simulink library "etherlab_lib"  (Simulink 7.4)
settings: Solver=ode45  SolverMode=SingleTasking  StartTime=0.0  StopTime=10.0  RelTol=1e-3
undefined symbols (not defined in the file or in its folder): ATD4, baumer_ecatencoder, bits, Boolean, BT, CoE, CW, DC, DI8DO8, Disabled, EK1100, EK1914, ekxxxx, EL1004, EL1262, EL1904, el1xxx, EL2004, EL2262, EL2535, el2535, EL2904, el2xxx, EL3002, EL3102, EL3201, EL3204, el320x_1, EL3255, EL3314, el331x, EL3356, el3356, EL3403, el3403, EL3602, el36x2, EL3702, el37x2, EL4002, el4xxx, EL5001, el500x, EL5021, el5021, EL5101, EL5152, El5152, EL51x1, el51xx, EL6001, el60xx, EL9110, el9xxx, EP1008, ep1xxx, EP2001, ep2xxx, EP3174, EP3182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
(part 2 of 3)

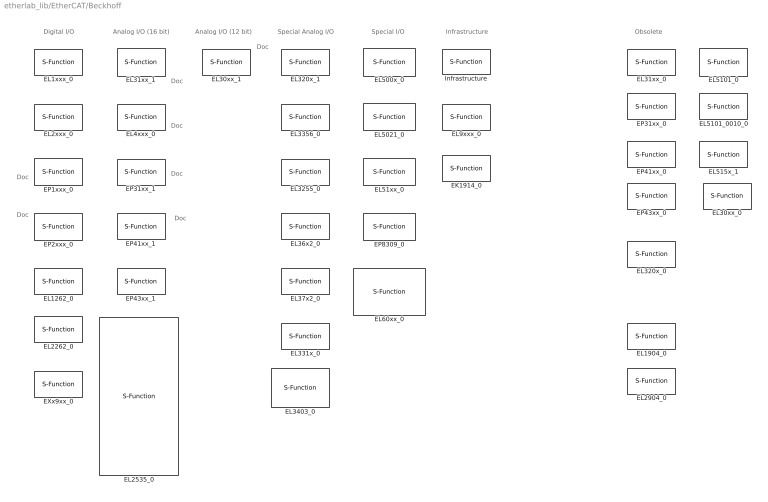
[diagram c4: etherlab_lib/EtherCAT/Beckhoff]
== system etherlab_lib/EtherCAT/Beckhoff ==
  note: Analog I/O (16 bit)
  note: Digital I/O
  note: Analog I/O (12 bit)
  note: Special Analog I/O
  note: Special I/O
  note: Infrastructure
  note: Obsolete
  note: Doc
  note: Doc
  note: Doc
  note: Doc
  note: Doc
  note: Doc
  note: Doc
  EK1914_0 : S-Function  FunctionName=ec_slave3  Parameters=Address,rv.SlaveConfig,rv.PortConfig,debug,tsample  SFunctionModules='ecrt_support'  EnableBusSupport=off  mask(EK1904){master=0, index=1, model=EK1914, stdio=on, safeio=off, tsample=-1, revision=, debug=}
      mask prompts: index "Slave Index"; model "Device Model"; stdio "Standard IO"; safeio "Safe IO"; tsample "Sample Time (-1 for inherited)"
      mask help: Beckhoff EtherCAT SAFE digital input/output coupler
      mask init:
      | Address = EtherCATSlave.formatAddress(master,index,tsample);
      | 
      | rv = ek1914(stdio, safeio);
      | 
      | rv.PortConfig.swap_io = EtherCATSlave.shouldSwapIoPorts();
      | 
      | text = sprintf('%s\\nM:%i Idx:%s', model, master, mat2str(index));
      | if numel(rv.PortConfig.input) > 1 || numel(rv.PortConfig.output) > 1
      |     EtherCATSlave.setPortNames(...
      |         {rv.PortConfig.input.portname},...
      |         {rv.PortConfig.output.portname});
      | 
      |     set_param(gcbh,'AttributesFormatString',text);
      | else
      |     set_param(gcbh,'AttributesFormatString','');
      |     set_param(gcbh,'MaskDisplay', strcat('disp(''',text,''')'));
      | end
  EL1262_0 : S-Function  FunctionName=ec_slave3  Parameters=Address,rv.SlaveConfig,rv.PortConfig,debug,tsample  SFunctionModules='ecrt_support'  EnableBusSupport=off  mask(EL1262){master=0, index=1, model=EL1262, one_ch=on, tsample=0, debug=0, revision=, dc_mode=10, dc_assign_activate=hex2dec('730'), dc_cycle0=0, dc_cycle0_factor=-10, dc_shift0=-10000, dc_shift0_factor=1, dc_shift0_input=off, dc_cycle1=0, dc_cycle1_factor=-1, dc_shift1=0, dc_shift1_factor=0}
      mask prompts: index "Slave Index"; model "Device Model"; one_ch "1 Ch. only"; tsample "Sample Time"; dc_mode "Mode/Oversampling"; dc_assign_activate "Assign Activate"; dc_cycle0 "Cycle Time Sync 0 [ns]"; dc_cycle0_factor "Factor"; dc_shift0 "Shift Time Sync0 [ns]"; dc_shift0_factor "Factor"; dc_shift0_input "Shift Time0 Input"; dc_cycle1 "Cycle Time Sync1 [ns]"; dc_cycle1_factor "Factor"; dc_shift1 "Shift Time Sync1 [ns]"; dc_shift1_factor "Factor"
      mask help: Beckhoff oversampling digital input
      mask init:
      | Address = EtherCATSlave.formatAddress(master,index,tsample);
      | 
      | rv = el1262(model).configure(one_ch,...
      |     [dc_mode, dc_assign_activate, ...
      |     dc_cycle0, dc_cycle0_factor,...
      |     dc_shift0, dc_shift0_factor, dc_shift0_input,...
      |     dc_cycle1, dc_cycle1_factor,...
      |     dc_shift1, dc_shift1_factor]);
      | rv.PortConfig.swap_io = EtherCATSlave.shouldSwapIoPorts();
  EL1904_0 : S-Function  FunctionName=ec_slave3  Parameters=Address,rv.SlaveConfig,rv.PortConfig,debug,tsample  SFunctionModules='ecrt_support'  EnableBusSupport=off  mask(EL1904){master=0, index=1, model=EL1904, safein=off, tsample=-1, revision=, debug=}
      mask prompts: index "Slave Index"; model "Device Model"; safein "Safe inputs"; tsample "Sample Time (-1 for inherited)"
      mask help: Beckhoff EtherCAT SAFE digital input
      mask init:
      | Address = EtherCATSlave.formatAddress(master,index,tsample);
      | 
      | rv = el1904(safein);
      | rv.PortConfig.swap_io = EtherCATSlave.shouldSwapIoPorts();
  EL1xxx_0 : S-Function  LoadFcn=el1xxx().checkModelName  FunctionName=ec_slave3  Parameters=Address,rv.SlaveConfig,rv.PortConfig,debug,tsample  SFunctionModules='ecrt_support'  EnableBusSupport=off  mask(EL1xxx){master=0, index=1, model=EL1004, revision=, vector=on, tsample=0, debug=0}
      mask prompts: index "Slave Index"; model "Device Model"; vector "Vector Outputs"; tsample "Sample Time"; debug "Debug Level"
      mask help: Beckhoff EtherCAT Digital Input
      mask init:
      | Address = EtherCATSlave.formatAddress(master,index,tsample);
      | 
      | rv = el1xxx(model).configure(vector);
      | rv.PortConfig.swap_io = EtherCATSlave.shouldSwapIoPorts();
  EL2262_0 : S-Function  FunctionName=ec_slave3  Parameters=Address,rv.SlaveConfig,rv.PortConfig,debug,tsample  SFunctionModules='ecrt_support'  EnableBusSupport=off  mask(EL2262){master=0, index=1, model=EL2262, one_ch=on, tsample=0, debug=0, revision=, dc_mode=10, dc_assign_activate=hex2dec('730'), dc_cycle0=0, dc_cycle0_factor=-10, dc_shift0=-10000, dc_shift0_factor=1, dc_shift0_input=off, dc_cycle1=0, dc_cycle1_factor=-1, dc_shift1=0, dc_shift1_factor=0}
      mask prompts: index "Slave Index"; model "Device Model"; one_ch "1 Ch. only"; tsample "Sample Time"; dc_mode "Mode/Oversampling"; dc_assign_activate "Assign Activate"; dc_cycle0 "Cycle Time Sync 0 [ns]"; dc_cycle0_factor "Factor"; dc_shift0 "Shift Time Sync0 [ns]"; dc_shift0_factor "Factor"; dc_shift0_input "Shift Time0 Input"; dc_cycle1 "Cycle Time Sync1 [ns]"; dc_cycle1_factor "Factor"; dc_shift1 "Shift Time Sync1 [ns]"; dc_shift1_factor "Factor"
      mask help: Beckhoff oversampling digital output
      mask init:
      | Address = EtherCATSlave.formatAddress(master,index,tsample);
      | 
      | rv = el2262(model).configure(one_ch,...
      |     [dc_mode, dc_assign_activate, ...
      |     dc_cycle0, dc_cycle0_factor,...
      |     dc_shift0, dc_shift0_factor, dc_shift0_input,...
      |     dc_cycle1, dc_cycle1_factor,...
      |     dc_shift1, dc_shift1_factor]);
      | rv.PortConfig.swap_io = EtherCATSlave.shouldSwapIoPorts();
  EL2535_0 : S-Function  LoadFcn=el2535().checkModelName  FunctionName=ec_slave3  Parameters=Address,rv.SlaveConfig,rv.PortConfig,debug,tsample  SFunctionModules='ecrt_support'  EnableBusSupport=off  mask(EL2535){master=0, index=1, model=EL2535, revision=, vector=on, tsample=0, debug=0, ch1enable=on, sdo_8=100, sdo_2=off, sdo_3=Default Value (see below), sdo_6=0, sdo_7=65535, sdo_9=350, sdo_10=6, sdo_11=50, sdo_1=off, sdo_12=100, sdo_13=10, ch2enable=on, sdo_23=100, sdo_17=off, sdo_18=Default Value (see below), sdo_21=0, sdo_22=65535, sdo_24=350, sdo_25=6, sdo_26=50, sdo_16=off, sdo_27=100, sdo_28=10, extra_output_1=None, extra_output_2=None, extra_output_3=None, extra_output_4=None}
      mask prompts: index "Slave Index"; model "Device Model"; vector "Vector Outputs"; tsample "Sample Time"; debug "Debug Level"; ch1enable "Enable"; sdo_8 "8000:10 - Maximum Current [%]"; sdo_2 "8000:04 - Invert Polarity"; sdo_3 "8000:05 - Watchdog"; sdo_6 "8000:0D - Default Output Value"; sdo_7 "8000:0E - Default Output Ramp"; sdo_9 "8000:12 - Current controller Kp"; sdo_10 "8000:13 - Current controller Ki"; sdo_11 "8000:14 - Current controller Kd"; sdo_1 "8000:03 - Enable dithering"; sdo_12 "8000:1E - Dithering Frequency [Hz]"; sdo_13 "8000:1F - Dithering Amplitude [% of max current in 8000:10]"; ch2enable "Enable"; sdo_23 "8010:10 - Maximum Current [%]"; sdo_17 "8010:04 - Invert Polarity"; sdo_18 "8010:05 - Watchdog"; sdo_21 "8010:0D - Default Output Value"; sdo_22 "8010:0E - Default Output Ramp"; sdo_24 "8010:12 - Current controller Kp"; sdo_25 "8010:13 - Current controller Ki"; sdo_26 "8010:14 - Current controller Kd"; sdo_16 "8010:03 - Enable dithering"; sdo_27 "8010:1E - Dithering Frequency [Hz]"; sdo_28 "8010:1F - Dithering Amplitude [% of max current in 8010:10]"; extra_output_1 "8000:21 - Extra Output 1"; extra_output_2 "8000:22 - Extra Output 2"; extra_output_3 "8010:21 - Extra Output 3"; extra_output_4 "8010:22 - Extra Output 4"
      mask help: Beckhoff EtherCAT PWM Output
      mask init:
      | Address = EtherCATSlave.formatAddress(master,index,tsample);
      | 
      | extra_output = [...
      |     extra_output_1,
      |     extra_output_2,
      |     extra_output_3,
      |     extra_output_4,
      | ];
      | channels = [ ...
      |     ch1enable; ...
      |     ch2enable; ...
      | ];
      | 
      |  sdo_4 = 0;
      |  sdo_5 = 65536;
      | sdo_19 = 0;
      | sdo_20 = 65536;
      | 
      | sdo_14 = el2535.extra_output_popup_sdo_map(extra_output_1);
      | sdo_15 = el2535.extra_output_popup_sdo_map(extra_output_2);
      | sdo_29 = el2535.extra_output_popup_sdo_map(extra_output_3);
      | sdo_30 = el2535.extra_output_popup_sdo_map(extra_output_4);
      | 
      | % fix watchdog value
      | sdo_3  =  sdo_3 - 1;
      | sdo_18 = sdo_18 - 1;
      | 
      | 
      | rv = el2535(model).configure(channels,extra_output, ...
      |     [  sdo_1,  sdo_2,  sdo_3,  sdo_4,  sdo_5,  sdo_6, ...
      |        sdo_7,  sdo_8,  sdo_9, sdo_10, sdo_11, sdo_12, ...
      |       sdo_13, sdo_14, sdo_15, sdo_16, sdo_17, sdo_18, ...
      |       sdo_19, sdo_20, sdo_21, sdo_22, sdo_23, sdo_24, ...
      |       sdo_25, sdo_26, sdo_27, sdo_28, sdo_29, sdo_30, ...
      |     ]);
      | 
      | rv.PortConfig.swap_io = EtherCATSlave.shouldSwapIoPorts();
      | 
      | inp = arrayfun(@(x) x.portname, rv.PortConfig.input, 'UniformOutput', false);
      | outp = arrayfun(@(x) x.portname, rv.PortConfig.output, 'UniformOutput', false);
      | 
      | if rv.OutputAmpere >= 1.0
      |     extra = sprintf('%s: %0.0f A', model, rv.OutputAmpere);
      | else
      |     extra = sprintf('%s: %0.0f mA', model, rv.OutputAmpere * 1000);
      | end
      | 
      | 
      | 
      | EtherCATSlave.setPortNames(inp, outp, extra);
      | 
      | set_param(gcb,'AttributesFormatString',...
      |     sprintf('%s\nM:%i Idx:%s',...
      |             extra,master,mat2str(index)))
  EL2904_0 : S-Function  FunctionName=ec_slave3  Parameters=Address,rv.SlaveConfig,rv.PortConfig,debug,tsample  SFunctionModules='ecrt_support'  EnableBusSupport=off  mask(EL2904){master=0, index=1, model=EL2904, safeout=off, tsample=-1, revision=, debug=}
      mask prompts: index "Slave Index"; model "Device Model"; safeout "Safe outputs"; tsample "Sample Time (-1 for inherited)"
      mask help: Beckhoff EtherCAT SAFE digital output
      mask init:
      | Address = EtherCATSlave.formatAddress(master,index,tsample);
      | 
      | rv = el2904(safeout);
      | rv.PortConfig.swap_io = EtherCATSlave.shouldSwapIoPorts();
  EL2xxx_0 : S-Function  LoadFcn=el2xxx().checkModelName  FunctionName=ec_slave3  Parameters=Address,rv.SlaveConfig,rv.PortConfig,debug,tsample  SFunctionModules='ecrt_support'  EnableBusSupport=off  mask(EL2xxx){master=0, index=1, model=EL2004, revision=, vector=on, diag=off, tsample=-1, debug=0}
      mask prompts: index "Slave Index"; model "Device Model"; vector "Vector Inputs"; diag "Diag Port"; tsample "Sample Time (-1 for inherited)"
      mask help: Beckhoff EtherCAT Digital Output
      mask init:
      | Address = EtherCATSlave.formatAddress(master,index,tsample);
      | 
      | rv = el2xxx(model).configure(vector,diag);
      | rv.PortConfig.swap_io = EtherCATSlave.shouldSwapIoPorts();
  EL30xx_0 : S-Function  LoadFcn=|  FunctionName=ec_slave3  Parameters=Address,rv.SlaveConfig,rv.PortConfig,debug,tsample  SFunctionModules='ecrt_support'  EnableBusSupport=off  mask(EL30xx){master=0, index=1, model=EL3002, vector=on, raw=off, scale=, offset=, tau=, tsample=0, debug=0}
      | el30xx('check')
      | if ~strcmp(bdroot(gcb),'etherlab_lib')
      |   disp([gcb ' is obsolete. Please replace'])
      | end
      mask prompts: index "Slave Index"; model "Device Model"; vector "Vector Output"; raw "Raw Bits"; scale "Output Scale"; offset "Output Offset"; tau "LPF Time Constant (sec)"; tsample "Sample Time"
      mask help: Beckhoff 1,2,4,8-Channel 16-Bit Analog Input
      mask init:
      | Address = EtherCATSlave.formatAddress(master,index,tsample);
      | 
      | el30xx('set');
      | 
      | rv = get_param(gcbh, 'UserData');
      | 
      | rv.PortConfig.swap_io = EtherCATSlave.shouldSwapIoPorts();
  EL30xx_1 : S-Function  LoadFcn=|  FunctionName=ec_slave3  Parameters=Address,rv.SlaveConfig,rv.PortConfig,debug,tsample  SFunctionModules='ecrt_support'  EnableBusSupport=off  mask(EL30xx){master=0, index=1, model=EL3002, revision=, vector=on, status=off, gain=[], offset=[], tau=[], tsample=0, debug=0, omega=, filter=Off, opmode=FreeRun, fastop=off}
      | el30xx_1().checkModelName()
      | EtherCATSlave.checkFilter()
      mask prompts: index "Slave Index"; model "Device Model"; vector "Vector Output"; status "Status Output"; gain "Output Scale"; offset "Output Offset"; tau "LPF time constant (s)"; tsample "Sample Time"; omega "deprecated"; opmode "Synchronization Mode (1C33:01.0)"; fastop "FastOp Mode (1C33:01.15)"
      mask help: Beckhoff 1,2,4,8-Channel 16-Bit Analog Input
      mask init:
      | Address = EtherCATSlave.formatAddress(master,index,tsample);
      | 
      | rv = el30xx_1(model).configure(status,vector,...
      |     EtherCATSlave.configureScale(2^15,gain,offset,tau),...
      |     [filter,opmode,fastop]);
      | 
      | rv.PortConfig.swap_io = EtherCATSlave.shouldSwapIoPorts();
      | 
      | if vector
      |     set_param(gcb,'AttributesFormatString','');
      | 
      |     set_param(gcb,'MaskDisplay',...
      |         sprintf('disp(''%s %s\\nM:%i Idx:%s'')',...
      |         model,rv.function,master,mat2str(index)))
      | else
      |     EtherCATSlave.setPortNames({},...
      |         {rv.PortConfig.output.portname})
      |     
      |     set_param(gcb,'AttributesFormatString',...
      |         sprintf('%s %s\nM:%i Idx:%s',...
      |         model,rv.function,master,mat2str(index)))
      | end
  EL31xx_0 : S-Function  LoadFcn=|  FunctionName=ec_slave3  Parameters=Address,rv.SlaveConfig,rv.PortConfig,debug,tsample  SFunctionModules='ecrt_support'  EnableBusSupport=off  mask(EL31xx){master=0, index=1, model=EL3102, dc=DC-Synchron, vector=on, raw=off, scale=, offset=, tau=, tsample=0, debug=0}
      | el31xx('check')
      | if ~strcmp(bdroot(gcb),'etherlab_lib')
      |   disp([gcb ' is obsolete. Please replace'])
      | end
      mask prompts: index "Slave Index"; model "Device Model"; dc "Distributed Clock"; vector "Vector Output"; raw "Raw output"; scale "Output Scale"; offset "Output Offset"; tau "LPF Time Constant (sec)"; tsample "Sample Time"
      mask help: Beckhoff 2,4,8-Channel 16-Bit Analog Input with Distributed Clocks Status output is not supported
      mask init:
      | Address = EtherCATSlave.formatAddress(master,index,tsample);
      | 
      | el31xx('set');  % Report errors
      | 
      | rv = get_param(gcb,'UserData');
      | rv.PortConfig.swap_io = EtherCATSlave.shouldSwapIoPorts();
  EL31xx_1 : S-Function  LoadFcn=|  FunctionName=ec_slave3  Parameters=Address,rv.SlaveConfig,rv.PortConfig,debug,tsample  SFunctionModules='ecrt_support'  EnableBusSupport=off  mask(EL31xx){master=0, index=1, model=EL3102, revision=, vector=on, status=off, filter=Off, gain=[], offset=[], tau=[], tsample=0, debug=0, omega=, dc_mode=Free Run/SM-Synchron, dc_assign_activate=hex2dec('700'), dc_cycle0=[], dc_cycle0_factor=[], dc_shift0=[], dc_shift0_factor=[], dc_shift0_input=off, dc_cycle1=[], dc_cycle1_factor=[], dc_shift1=[], dc_shift1_factor=[]}
      | el31xx_1().checkModelName()
      | EtherCATSlave.checkFilter()
      mask prompts: index "Slave Index"; model "Device Model"; vector "Vector Output"; status "Status output"; gain "Output Gain"; offset "Output Offset"; tau "LPF time constant (s)"; tsample "Sample Time"; omega "deprecated"; dc_mode "Mode"; dc_assign_activate "Assign Activate"; dc_cycle0 "Cycle Time Sync 0"; dc_cycle0_factor "Factor"; dc_shift0 "Shift Time Sync0"; dc_shift0_factor "Factor"; dc_shift0_input "Shift Time0 Input"; dc_cycle1 "Cycle Time Sync1"; dc_cycle1_factor "Factor"; dc_shift1 "Shift Time Sync1"; dc_shift1_factor "Factor"
      mask help: Beckhoff 2,4,8-Channel 16-Bit Analog Input with Distributed Clocks
      mask init:
      | Address = EtherCATSlave.formatAddress(master,index,tsample);
      | 
      | rv = el31xx_1(model).configure(status,vector,...
      |     EtherCATSlave.configureScale(2^15,gain,offset,tau),...
      |     [dc_mode, dc_assign_activate, ...
      |      dc_cycle0, dc_cycle0_factor, ...
      |      dc_shift0, dc_shift0_factor, dc_shift0_input, ...
      |      dc_cycle1, dc_cycle1_factor, ...
      |      dc_shift1, dc_shift1_factor], ...
      |      filter);
      | 
      | rv.PortConfig.swap_io = EtherCATSlave.shouldSwapIoPorts();
      | 
      | if vector || model(6) == '1'
      |     set_param(gcb,'AttributesFormatString','');
      | 
      |     set_param(gcb,'MaskDisplay',...
      |         sprintf('disp(''%s\\nM:%i Idx:%s'')',...
      |         model,master,mat2str(index)))
      | else
      |     EtherCATSlave.setPortNames({},...
      |         {rv.PortConfig.output.portname})
      |     
      |     set_param(gcb,'AttributesFormatString',...
      |         sprintf('%s\nM:%i Idx:%s',...
      |         model,master,mat2str(index)))
      | end
  EL320x_0 : S-Function  LoadFcn=|  FunctionName=ec_slave3  Parameters=Address,rv.SlaveConfig,rv.PortConfig,debug,tsample  SFunctionModules='ecrt_support'  EnableBusSupport=off  mask(EL320x){master=0, index=1, model=EL3204, rtd=0, technology=2, filter=50 Hz, vector=on, enable_status=on, tsample=0, debug=0}
      | el320x('check')
      | if ~strcmp(bdroot(gcb),'etherlab_lib')
      |   disp([gcb ' is obsolete. Please replace'])
      | end
      mask prompts: index "Slave Index"; model "Device Model"; rtd "RTD-Element (CoE 80x0:19)"; technology "Connection Technology (CoE 80x0:1A)"; filter "Filter (CoE 8000:15)"; vector "Vector Output"; enable_status "Status Port"; tsample "Sample Time"
      mask help: Beckhoff 1, 2, 4-Channel Input Terminal Pt100 (RTD)
      mask init:
      | Address = EtherCATSlave.formatAddress(master,index,tsample);
      | 
      | SdoConfig = [];
      | 
      | rv = get_param(gcbh,'UserData');
      | 
      | count = numel(rv.SlaveConfig.sm{1}{3});
      | 
      | err = {};
      | if numel(rtd) == 1
      |     rtd = repmat(rtd,1,count);
      | elseif numel(rtd) ~= count
      |     err = {['- Mask option "RTD Element"' ...
      |         ' is not a scalar or vector with ' ...
      |         num2str(count) ' elements']};
      | end
      | 
      | if numel(technology) == 1
      |     technology = repmat(technology,1,count);
      | elseif numel(technology) ~= count
      |     err = horzcat(err, ['- Mask option "Connection Technology"' ...
      |         ' is not a scalar or vector with ' ...
      |         num2str(count) ' elements']);
      | end
      | 
      | if ~isempty(err)
      |     errordlg(err,gcb);
      |     return
      | end
      | 
      | rv.SlaveConfig.sdo = num2cell(vertcat(...
      |     [hex2dec('8000'),6,8,1],...
      |     [hex2dec('8000'),hex2dec('15'),16,filter+1],...
      |     horzcat(repmat(hex2dec('8000') + 16*(0:count-1)',2,1),...
      |             [hex2dec('19')*ones(count,1);hex2dec('1a')*ones(count,1)],...
      |             16*ones(count*2,1),...
      |             vertcat(reshape(rtd,[],1),...
      |                     reshape(technology,[],1)))));
      | 
      | rv.PortConfig.swap_io = EtherCATSlave.shouldSwapIoPorts();
  EL320x_1 : S-Function  LoadFcn=el320x_1().checkModelName()  FunctionName=ec_slave3  Parameters=Address,rv.SlaveConfig,rv.PortConfig,debug,tsample  SFunctionModules='ecrt_support'  EnableBusSupport=off  mask(EL320x){master=0, index=1, model=EL3201, revision=, filter=Off, vector=on, status=off, tsample=0, debug=0, sdo_01=Pt100 -200...850C, sdo_02=2-wire, sdo_03=0, sdo_04=Pt100 -200...850C, sdo_05=2-wire, sdo_06=0, sdo_07=Pt100 -200...850C, sdo_08=2-wire, sdo_09=0, sdo_10=Pt100 -200...850C, sdo_11=2-wire, sdo_12=0, sdo_13=Pt100 -200...850C, sdo_14=2-wire, sdo_15=0, sdo_16=Pt100 -200...850C, sdo_17=2-wire, sdo_18=0, sdo_19=Pt100 -200...850C, sdo_20=2-wire, sdo_21=0, sdo_22=Pt100 -200...850C, sdo_23=2-wire, sdo_24=0}
      mask prompts: index "Slave Index"; model "Device Model"; vector "Vector Output"; status "Status Port"; tsample "Sample Time"; sdo_01 "RTD-Element"; sdo_02 "Technology"; sdo_03 "Wire Calibration (1/32 Ohm)"; sdo_04 "RTD-Element"; sdo_05 "Technology"; sdo_06 "Wire Calibration (1/32 Ohm)"; sdo_07 "RTD-Element"; sdo_08 "Technology"; sdo_09 "Wire Calibration (1/32 Ohm)"; sdo_10 "RTD-Element"; sdo_11 "Technology"; sdo_12 "Wire Calibration (1/32 Ohm)"; sdo_13 "RTD-Element"; sdo_14 "Technology"; sdo_15 "Wire Calibration (1/32 Ohm)"; sdo_16 "RTD-Element"; sdo_17 "Technology"; sdo_18 "Wire Calibration (1/32 Ohm)"; sdo_19 "RTD-Element"; sdo_20 "Technology"; sdo_21 "Wire Calibration (1/32 Ohm)"; sdo_22 "RTD-Element"; sdo_23 "Technology"; sdo_24 "Wire Calibration (1/32 Ohm)"
      mask help: Beckhoff 1, 2, 4-Channel Input Terminal Pt100 (RTD)
      mask init:
      | Address = EtherCATSlave.formatAddress(master,index,tsample);
      | 
      | rv = el320x_1(model).configure(status,vector,filter,...
      |     [sdo_01,sdo_04,sdo_07,sdo_10,sdo_13,sdo_16,sdo_19,sdo_22] - 1,...
      |     [sdo_02,sdo_05,sdo_08,sdo_11,sdo_14,sdo_17,sdo_20,sdo_23] - 1,...
      |     [sdo_03,sdo_06,sdo_09,sdo_12,sdo_15,sdo_18,sdo_21,sdo_24]);
      | 
      | rv.PortConfig.swap_io = EtherCATSlave.shouldSwapIoPorts();
      | 
      | if vector || model(6) == '1'
      |     set_param(gcb,'AttributesFormatString','');
      | 
      |     set_param(gcb,'MaskDisplay',...
      |         sprintf('disp(''%s\\nM:%i Idx:%s'')',...
      |         model,master,mat2str(index)))
      | else
      |     EtherCATSlave.setPortNames({},...
      |         {rv.PortConfig.output.portname})
      |     
      |     set_param(gcb,'AttributesFormatString',...
      |         sprintf('%s\nM:%i Idx:%s',...
      |         model,master,mat2str(index)))
      | end
  EL3255_0 : S-Function  LoadFcn=|  FunctionName=ec_slave3  Parameters=Address,rv.SlaveConfig,rv.PortConfig,debug,tsample  SFunctionModules='ecrt_support'  EnableBusSupport=off  mask(EL3255){master=0, index=1, model=EL3255, revision=, channels=1, vector=off, gain=[], offset=[], tau=[], tsample=0, debug=0, omega=, dc_mode=Free Run/SM-Synchron, dc_assign_activate=hex2dec('700'), dc_cycle0=[], dc_cycle0_factor=[], dc_shift0=[], dc_shift0_factor=[], dc_shift0_input=off, dc_cycle1=[], dc_cycle1_factor=[], dc_shift1=[], dc_shift1_factor=[], sdo_01=off, sdo_02=50 Hz, sdo_03=Off (up to 10 kOhm), sdo_04=Off (up to 10 kOhm), sdo_05=Off (up to 10 kOhm), sdo_06=Off (up to 10 kOhm), sdo_07=Off (up to 10 kOhm)}
      | el3255().checkModelName()
      | EtherCATSlave.checkFilter
      mask prompts: index "Slave Index"; model "Device Model"; channels "Active Channels"; vector "Vector Outputs"; tau "LPF time constant (s)"; tsample "Sample Time"; debug "Debug Level"; omega "deprecated"; dc_mode "Distributed Clock"; dc_assign_activate "Assign Activate"; dc_cycle0 "Cycle Time Sync 0"; dc_cycle0_factor "Factor"; dc_shift0 "Shift Time Sync0"; dc_shift0_factor "Factor"; dc_shift0_input "Shift Time0 Input"; dc_cycle1 "Cycle Time Sync1"; dc_cycle1_factor "Factor"; dc_shift1 "Shift Time Sync1"; dc_shift1_factor "Factor"; sdo_01 "Enable Filter (#x8000:06)"; sdo_02 "Filter settings (#x8000:15)"; sdo_03 "Load resistance 1"; sdo_04 "Load resistance 2"; sdo_05 "Load resistance 3"; sdo_06 "Load resistance 4"; sdo_07 "Load resistance 5"
      mask help: Beckhoff EtherCAT 5Ch. potentiometer measurement with sensor supply
      mask init:
      | Address = EtherCATSlave.formatAddress(master,index,tsample);
      | 
      | rv = el3255(model).configure(channels,vector,...
      |     [dc_mode, dc_assign_activate, ...
      |     dc_cycle0, dc_cycle0_factor,...
      |     dc_shift0, dc_shift0_factor, dc_shift0_input,...
      |     dc_cycle1, dc_cycle1_factor,...
      |     dc_shift1, dc_shift1_factor], ...
      |     EtherCATSlave.configureScale(2^15,gain,offset,tau),...
      |     [sdo_01, ...
      |      [sdo_02, sdo_03, sdo_04, sdo_05, sdo_06, sdo_07]-1]);
      | 
      | rv.PortConfig.swap_io = EtherCATSlave.shouldSwapIoPorts();
  EL331x_0 : S-Function  LoadFcn=el331x().checkModelName  FunctionName=ec_slave3  Parameters=Address,rv.SlaveConfig,rv.PortConfig,debug,tsample  SFunctionModules='ecrt_support'  EnableBusSupport=off  mask(EL331x){master=0, index=1, model=EL3314, revision=, vector=on, status=off, tsample=0, debug=0, sdo_8000_02=0.1, sdo_8000_0C=Internal, sdo_8000_15=50 Hz, sdo_8000_19=0: Type K, sdo_8000_1A=Inactive, sdo_8010_02=0.1, sdo_8010_0C=Internal, sdo_8010_15=50 Hz, sdo_8010_19=0: Type K, sdo_8010_1A=Inactive, sdo_8020_02=0.1, sdo_8020_0C=Internal, sdo_8020_15=50 Hz, sdo_8020_19=0: Type K, sdo_8020_1A=Inactive, sdo_8030_02=0.1, sdo_8030_0C=Internal, sdo_8030_15=50 Hz, sdo_8030_19=0: Type K, sdo_8030_1A=Inactive, sdo_8040_02=0.1, sdo_8040_0C=Internal, sdo_8040_15=50 Hz, sdo_8040_19=0: Type K, sdo_8040_1A=Inactive, sdo_8050_02=0.1, sdo_8050_0C=Internal, sdo_8050_15=50 Hz, sdo_8050_19=0: Type K, sdo_8050_1A=Inactive, sdo_8060_02=0.1, sdo_8060_0C=Internal, sdo_8060_15=50 Hz, sdo_8060_19=0: Type K, sdo_8060_1A=Inactive, sdo_8070_02=0.1, sdo_8070_0C=Internal, sdo_8070_15=50 Hz, sdo_8070_19=0: Type K, sdo_8070_1A=Inactive}
      mask prompts: index "Slave Index"; model "Device Model"; vector "Vector Outputs"; status "Status Output"; tsample "Sample Time"; sdo_8000_02 "Resolution (#x8000:02)"; sdo_8000_0C "Coldjunction Compensation (#x8000:0C)"; sdo_8000_15 "Filter settings (#x8000:15)"; sdo_8000_19 "TC Element (#x8000:19)"; sdo_8000_1A "MC Filter (#x8000:1A)"; sdo_8010_02 "Resolution (#x8010:02)"; sdo_8010_0C "Coldjunction Compensation (#x8010:0C)"; sdo_8010_15 "Filter settings (#x8010:15)"; sdo_8010_19 "TC Element (#x8010:19)"; sdo_8010_1A "MC Filter (#x8010:1A)"; sdo_8020_02 "Resolution (#x8020:02)"; sdo_8020_0C "Coldjunction Compensation (#x8020:0C)"; sdo_8020_15 "Filter settings (#x8020:15)"; sdo_8020_19 "TC Element (#x8020:19)"; sdo_8020_1A "MC Filter (#x8020:1A)"; sdo_8030_02 "Resolution (#x8030:02)"; sdo_8030_0C "Coldjunction Compensation (#x8030:0C)"; sdo_8030_15 "Filter settings (#x8030:15)"; sdo_8030_19 "TC Element (#x8030:19)"; sdo_8030_1A "MC Filter (#x8030:1A)"; sdo_8040_02 "Resolution (#x8040:02)"; sdo_8040_0C "Coldjunction Compensation (#x8040:0C)"; sdo_8040_15 "Filter settings (#x8040:15)"; sdo_8040_19 "TC Element (#x8040:19)"; sdo_8040_1A "MC Filter (#x8040:1A)"; sdo_8050_02 "Resolution (#x8050:02)"; sdo_8050_0C "Coldjunction Compensation (#x8050:0C)"; sdo_8050_15 "Filter settings (#x8050:15)"; sdo_8050_19 "TC Element (#x8050:19)"; sdo_8050_1A "MC Filter (#x8050:1A)"; sdo_8060_02 "Resolution (#x8060:02)"; sdo_8060_0C "Coldjunction Compensation (#x8060:0C)"; sdo_8060_15 "Filter settings (#x8060:15)"; sdo_8060_19 "TC Element (#x8060:19)"; sdo_8060_1A "MC Filter (#x8060:1A)"; sdo_8070_02 "Resolution (#x8070:02)"; sdo_8070_0C "Coldjunction Compensation (#x8070:0C)"; sdo_8070_15 "Filter settings (#x8070:15)"; sdo_8070_19 "TC Element (#x8070:19)"; sdo_8070_1A "MC Filter (#x8070:1A)"
      mask help: Beckhoff thermocouple input slave terminal
      mask init:
      | Address = EtherCATSlave.formatAddress(master,index,tsample);
      | 
      | rv = el331x(model).configure(vector,status,...
      |     [sdo_8000_02,sdo_8000_0C,sdo_8000_15,sdo_8000_19,sdo_8000_1A;
      |      sdo_8010_02,sdo_8010_0C,sdo_8010_15,sdo_8010_19,sdo_8010_1A;
      |      sdo_8020_02,sdo_8020_0C,sdo_8020_15,sdo_8020_19,sdo_8020_1A;
      |      sdo_8030_02,sdo_8030_0C,sdo_8030_15,sdo_8030_19,sdo_8030_1A;
      |      sdo_8040_02,sdo_8040_0C,sdo_8040_15,sdo_8040_19,sdo_8040_1A;
      |      sdo_8050_02,sdo_8050_0C,sdo_8050_15,sdo_8050_19,sdo_8050_1A;
      |      sdo_8060_02,sdo_8060_0C,sdo_8060_15,sdo_8060_19,sdo_8060_1A;
      |      sdo_8070_02,sdo_8070_0C,sdo_8070_15,sdo_8070_19,sdo_8070_1A]);
      | 
      | rv.PortConfig.swap_io = EtherCATSlave.shouldSwapIoPorts();
  EL3356_0 : S-Function  LoadFcn=el3356().checkModelName()  FunctionName=ec_slave3  Parameters=Address,rv.SlaveConfig,rv.PortConfig,debug,tsample  SFunctionModules='ecrt_support'  EnableBusSupport=off  mask(EL3356){master=0, index=1, model=EL3356, revision=, adc=off, range=[], scale=[], offset=[], tau=[], tsample=-1, debug=0, omega=, dc_mode=SM-Synchron, dc_assign_activate=hex2dec('320'), dc_cycle0=0, dc_cycle0_factor=1, dc_shift0=0, dc_shift0_factor=0, dc_shift0_input=off, dc_cycle1=0, dc_cycle1_factor=1, dc_shift1=0, dc_shift1_factor=0, sdo_01=off, sdo_02=off, sdo_03=on, sdo_04=on, sdo_05=off, sdo_06=FIR 50 Hz, sdo_07=FIR 50 Hz, sdo_08=10, sdo_09=20, sdo_10=1000, sdo_11=5, sdo_12=1800, sdo_13=10, sdo_14=off, sdo_15=50 Hz FIR, sdo_16=off, sdo_17=50 Hz FIR}
      mask prompts: index "Slave Index"; model "Device Model"; adc "2 ch ADC only"; range "RMB Range [mV/V]"; scale "Output Scale"; offset "Output Offset"; tau "LPF time constant (s)"; tsample "Sample Time"; omega "deprecated"; dc_mode "Mode"; dc_assign_activate "Assign Activate"; dc_cycle0 "Cycle Time Sync 0"; dc_cycle0_factor "Factor"; dc_shift0 "Shift Time Sync0"; dc_shift0_factor "Factor"; dc_shift0_input "Shift Time0 Input"; dc_cycle1 "Cycle Time Sync1"; dc_cycle1_factor "Factor"; dc_shift1 "Shift Time Sync1"; dc_shift1_factor "Factor"; sdo_01 "Mode 0 Enable Filter (#x8000:01)"; sdo_02 "Mode 1 Enable Filter (#x8000:02)"; sdo_03 "Mode 0 Enable Averager (#x8000:03)"; sdo_04 "Mode 1 Enable Averager (#x8000:04)"; sdo_05 "Symmetric Reference Potential (#x8000:05)"; sdo_06 "Mode 0 Filter (#x8000:11)"; sdo_07 "Mode 1 Filter (#x8000:12)"; sdo_08 "Dynamic filter change time [0.01s] (#x8000:13)"; sdo_09 "Dynamic filter delta (#x8000:14)"; sdo_10 "Steady state window (#x8000:29)"; sdo_11 "Steady state tolerance (#x8000:2a)"; sdo_12 "Calibration interval [100ms] (#x8000:31)"; sdo_13 "Test interval (#x8000:32)"; sdo_14 "Enable ch. 1 filter (#x8010:06)"; sdo_15 "Ch.1 filter settings (#x8010:15)"; sdo_16 "Enable ch.2 filter (#x8020:06)"; sdo_17 "Ch.2 filter settings (#x8020:15)"
      mask help: Beckhoff DMS Input with Distributed Clocks
      mask init:
      | Address = EtherCATSlave.formatAddress(master,index,tsample);
      | 
      | rv = el3356(model).configure(adc,range,...
      |     [dc_mode, dc_assign_activate, ...
      |     dc_cycle0, dc_cycle0_factor,...
      |     dc_shift0, dc_shift0_factor, dc_shift0_input,...
      |     dc_cycle1, dc_cycle1_factor,...
      |     dc_shift1, dc_shift1_factor], ...
      |     EtherCATSlave.configureScale(2^31,scale,offset,tau),...
      |     [sdo_01,   sdo_02,   sdo_03, sdo_04, sdo_05, ...
      |      sdo_06-1, sdo_07-1, sdo_08, sdo_09, sdo_10, ...
      |      sdo_11,   sdo_12,   sdo_13, ...
      |      sdo_14,   sdo_15-1, ...
      |      sdo_16,   sdo_17-1]);
      | 
      | rv.PortConfig.swap_io = EtherCATSlave.shouldSwapIoPorts();
      | 
      | EtherCATSlave.setPortNames(...
      |     {rv.PortConfig.input.portname},...
      |     {rv.PortConfig.output.portname});
      | 
      | set_param(gcb,'AttributesFormatString',...
      |     sprintf('%s\nM:%i Idx:%s',...
      |             model,master,mat2str(index)))
  EL3403_0 : S-Function  LoadFcn=el3403().checkModelName()  FunctionName=ec_slave3  Parameters=Address,rv.SlaveConfig,rv.PortConfig,debug,tsample  SFunctionModules='ecrt_support'  EnableBusSupport=off  mask(EL3403){master=0, index=1, model=EL3403, variant=off, current=1, voltage=1, tsample=-1, revision=[223031378 1441792], debug=0, freq=Phase L1, ref=Phase L1, zerocross=5, cycle=10}
      mask prompts: index "Slave Index"; model "Device Model"; variant "Variants"; current "Current Transformation Ratio 1:"; voltage "Voltage Transformation Ratio 1:"; tsample "Sample Time (-1 inherited)"; freq "Frequency channel (F800:05)"; ref "Reference channel (F800:0E)"; zerocross "Zero cross timeout (F800:21)"; cycle "Line cycle (F800:22)"
      mask help: Beckhoff 3-phase power measurement terminal
      mask init:
      | Address = EtherCATSlave.formatAddress(master,index,tsample);
      | 
      | rv = el3403(model).configure(variant,current,voltage,...
      |     [freq-1, ref-1, zerocross, cycle]);
      | 
      | rv.PortConfig.swap_io = EtherCATSlave.shouldSwapIoPorts();
      | 
      | EtherCATSlave.setPortNames(...
      |     {rv.PortConfig.input.portname},...
      |     {rv.PortConfig.output.portname});
      | 
      | set_param(gcb,'AttributesFormatString',...
      |     sprintf('%s\nM:%i Idx:%s',...
      |             model,master,mat2str(index)))
  EL36x2_0 : S-Function  LoadFcn=el36x2().checkModelName()  FunctionName=ec_slave3  Parameters=Address,rv.SlaveConfig,rv.PortConfig,debug,tsample,rv.Parameter,scale,offset  SFunctionModules='ecrt_support'  EnableBusSupport=off  mask(EL36x2){master=0, index=1, model=EL3602, revision=, vector=on, status=off, one_ch=on, scale=[], offset=[], tsample=0, debug=, sdo_x8000_15=50 Hz, sdo_x8000_19=+/- 10 V, sdo_x8010_19=+/- 10 V}
      mask prompts: index "Slave Index"; model "Device Model"; vector "Vector Output"; status "Status port"; one_ch "1 Ch. only"; scale "Output Scale"; offset "Output Offset"; tsample "Sample Time"; sdo_x8000_15 "Filter (#x8000:15)"; sdo_x8000_19 "Range Ch.1 (#x8000:19)"; sdo_x8010_19 "Range Ch.2 (#x8010:19)"
      mask help: Beckhoff 24-bit analog input terminal
      mask init:
      | Address = EtherCATSlave.formatAddress(master,index,tsample);
      | 
      | rv = el36x2(model).configure(one_ch,vector,status,...
      |     [numel(scale), 6; numel(offset), 7],...
      |     sdo_x8000_15-1,...
      |     [sdo_x8000_19,sdo_x8010_19]-1);
      | 
      | rv.PortConfig.swap_io = EtherCATSlave.shouldSwapIoPorts();
      | 
      | if ~status || vector || model(6) == '1' || one_ch
      |     set_param(gcb,'AttributesFormatString','');
      | 
      |     set_param(gcb,'MaskDisplay',...
      |         sprintf('disp(''%s\\nM:%i Idx:%s'')',...
      |         model,master,mat2str(index)))
      | else
      |     EtherCATSlave.setPortNames({},...
      |         {rv.PortConfig.output.portname})
      |     
      |     set_param(gcb,'AttributesFormatString',...
      |         sprintf('%s\nM:%i Idx:%s',...
      |         model,master,mat2str(index)))
      | end
  EL37x2_0 : S-Function  LoadFcn=el37x2().checkModelName()  FunctionName=ec_slave3  Parameters=Address,rv.SlaveConfig,rv.PortConfig,debug,tsample  SFunctionModules='ecrt_support'  EnableBusSupport=off  mask(EL37x2){master=0, index=1, model=EL3702, revision=, one_ch=off, scale=[], offset=[], tsample=0, debug=0, dc_mode=10, dc_assign_activate=hex2dec('730'), dc_cycle0=0, dc_cycle0_factor=-10     % 10-times OS, dc_shift0=-10000, dc_shift0_factor=1, dc_shift0_input=off, dc_cycle1=0, dc_cycle1_factor=-1, dc_shift1=0, dc_shift1_factor=0}
      mask prompts: index "Slave Index"; model "Device Model"; one_ch "1 Ch. only"; scale "Output Scale"; offset "Output Offset"; tsample "Sample Time"; dc_mode "Mode/Oversampling"; dc_assign_activate "Assign Activate"; dc_cycle0 "Cycle Time Sync 0 [ns]"; dc_cycle0_factor "Factor"; dc_shift0 "Shift Time Sync0 [ns]"; dc_shift0_factor "Factor"; dc_shift0_input "Shift Time0 Input"; dc_cycle1 "Cycle Time Sync1 [ns]"; dc_cycle1_factor "Factor"; dc_shift1 "Shift Time Sync1 [ns]"; dc_shift1_factor "Factor"
      mask help: Beckhoff oversampling analog input
      mask init:
      | Address = EtherCATSlave.formatAddress(master,index,tsample);
      | 
      | rv = el37x2(model).configure(one_ch,...
      |     [dc_mode, dc_assign_activate, ...
      |     dc_cycle0, dc_cycle0_factor,...
      |     dc_shift0, dc_shift0_factor, dc_shift0_input,...
      |     dc_cycle1, dc_cycle1_factor,...
      |     dc_shift1, dc_shift1_factor], ...
      |     EtherCATSlave.configureScale(2^15,scale,offset));
      | 
      | rv.PortConfig.swap_io = EtherCATSlave.shouldSwapIoPorts();
  EL4xxx_0 : S-Function  LoadFcn=el4xxx().checkModelName()  FunctionName=ec_slave3  Parameters=Address,rv.SlaveConfig,rv.PortConfig,debug,tsample  SFunctionModules='ecrt_support'  EnableBusSupport=off  mask(EL4xxx){master=0, index=1, model=EL4002, revision=, vector=on, scale=[], tsample=-1, debug=0, dc_mode=Free Run, dc_assign_activate=hex2dec('700'), dc_cycle0=0, dc_cycle0_factor=1, dc_shift0=0, dc_shift0_factor=0, dc_shift0_input=off, dc_cycle1=0, dc_cycle1_factor=1, dc_shift1=10000, dc_shift1_factor=0}
      mask prompts: index "Slave Index"; model "Device Model"; vector "Vector Input"; scale "Input Scale (empty for none)"; tsample "Sample Time (-1 for inherited)"; dc_mode "Distributed Clocks"; dc_assign_activate "Assign Activate"; dc_cycle0 "Cycle Time Sync 0"; dc_cycle0_factor "Factor"; dc_shift0 "Shift Time Sync0"; dc_shift0_factor "Factor"; dc_shift0_input "Shift Time0 Input"; dc_cycle1 "Cycle Time Sync1"; dc_cycle1_factor "Factor"; dc_shift1 "Shift Time Sync1"; dc_shift1_factor "Factor"
      mask help: Beckhoff Analog Output
      mask init:
      | Address = EtherCATSlave.formatAddress(master,index,tsample);
      | 
      | rv = el4xxx(model).configure(vector,...
      |     EtherCATSlave.configureScale(2^15,scale),...
      |     [dc_mode, dc_assign_activate,...
      |      dc_cycle0, dc_cycle0_factor,...
      |      dc_shift0, dc_shift0_factor, dc_shift0_input,...
      |      dc_cycle1, dc_cycle1_factor,...
      |      dc_shift1, dc_shift1_factor]);
      | 
      | rv.PortConfig.swap_io = EtherCATSlave.shouldSwapIoPorts();
  EL500x_0 : S-Function  LoadFcn=el500x().checkModelName()  FunctionName=ec_slave3  Parameters=Address,rv.SlaveConfig,rv.PortConfig,debug,tsample  SFunctionModules='ecrt_support'  EnableBusSupport=off  mask(EL500x){master=0, index=1, model=EL5001, revision=, pdo_x1A02=off, tsample=0, debug=0, dc_mode=FreeRun/SM-Synchron, dc_assign_activate=hex2dec('700')    % '120' for EL5001-0011, dc_cycle0=0, dc_cycle0_factor=1, dc_shift0=0, dc_shift0_factor=0, dc_shift0_input=off, dc_cycle1=0, dc_cycle1_factor=1, dc_shift1=15000, dc_shift1_factor=0, sdo_01=off, sdo_02=off, sdo_03=off, sdo_04=off, sdo_05=off, sdo_06=Gray, sdo_07=500k, sdo_08=Multiturn (25 bits), sdo_09=25, sdo_10=24, sdo_11=0, sdo_12=off, sdo_13=off, sdo_14=off, sdo_15=off, sdo_16=Gray, sdo_17=500k, sdo_18=Multiturn (25 bits), sdo_19=25, sdo_20=24, sdo_21=0}
      mask prompts: index "Slave Index"; model "Device Model"; pdo_x1A02 "Timestamp (PDO #x1a02)"; tsample "Sample Time"; dc_mode "DC Mode"; dc_assign_activate "Assign Activate"; dc_cycle0 "Cycle Time Sync 0 [ns]"; dc_cycle0_factor "Factor"; dc_shift0 "Shift Time Sync0 [ns]"; dc_shift0_factor "Factor"; dc_shift0_input "Shift Time0 Input"; dc_cycle1 "Cycle Time Sync1 [ns]"; dc_cycle1_factor "Factor"; dc_shift1 "Shift Time Sync1 [ns]"; dc_shift1_factor "Factor"; sdo_01 "8000:01 - Disable frame error"; sdo_02 "8000:02 - Enable power failure bit"; sdo_03 "8000:03 - Enable inhibit time"; sdo_04 "8000:04 - Enable test mode"; sdo_05 "8000:05 - Check SSI-frame size"; sdo_06 "8000:06 - SSI-coding"; sdo_07 "8000:09 - SSI-baudrate"; sdo_08 "8000:0F - SSI-frame type"; sdo_09 "8000:11 - SSI-frame size"; sdo_10 "8000:12 - SSI-data length"; sdo_11 "8000:13 - Min Inhibit Time [us]"; sdo_12 "8010:01 - Disable frame error"; sdo_13 "8010:02 - Enable power failure bit"; sdo_14 "8010:03 - Enable inhibit time"; sdo_15 "8010:04 - Enable test mode"; sdo_16 "8010:06 - SSI-coding"; sdo_17 "8010:09 - SSI-baudrate"; sdo_18 "8010:0F - SSI-frame type"; sdo_19 "8010:11 - SSI-frame size"; sdo_20 "8010:12 - SSI-data length"; sdo_21 "8010:13 - Min Inhibit Time [us]"
      mask help: Beckhoff EtherCAT SSI Input
      mask init:
      | Address = EtherCATSlave.formatAddress(master,index,tsample);
      | 
      | rv = el500x(model).configure(pdo_x1A02, ...
      |     [  sdo_01,   sdo_02, sdo_03,   sdo_04,   sdo_05, sdo_06-1,...
      |      sdo_07-1, sdo_08-1, sdo_09,   sdo_10,   sdo_11,   sdo_12,...
      |        sdo_13,   sdo_14, sdo_15, sdo_16-1, sdo_17-1, sdo_18-1,...
      |        sdo_19,   sdo_20, sdo_21],...
      |     [dc_mode, dc_assign_activate, ...
      |      dc_cycle0, dc_cycle0_factor,...
      |      dc_shift0, dc_shift0_factor, dc_shift0_input,...
      |      dc_cycle1, dc_cycle1_factor,...
      |      dc_shift1, dc_shift1_factor]);
      | 
      | rv.PortConfig.swap_io = EtherCATSlave.shouldSwapIoPorts();
      | 
      | if numel(rv.PortConfig.output) > 2
      |     EtherCATSlave.setPortNames({},...
      |         {rv.PortConfig.output.portname});
      |     
      |     set_param(gcb,'AttributesFormatString',...
      |         sprintf('%s\nM:%i Idx:%s',...
      |         model,master,mat2str(index)))
      | else
      |     set_param(gcb,'AttributesFormatString','');
      | 
      |     set_param(gcb,'MaskDisplay',...
      |         sprintf('disp(''%s\\nM:%i Idx:%s'')',...
      |         model,master,mat2str(index)))
      | end
  EL5021_0 : S-Function  LoadFcn=el5021().checkModelName()  FunctionName=ec_slave3  Parameters=Address,rv.SlaveConfig,rv.PortConfig,debug,tsample  SFunctionModules='ecrt_support'  EnableBusSupport=off  mask(EL5021){master=0, index=1, model=EL5021, revision=, tsample=-1, debug=0, dc_mode=FreeRun/SM-Synchron, dc_assign_activate=hex2dec('700'), dc_cycle0=0, dc_cycle0_factor=1, dc_shift0=-30600, dc_shift0_factor=0, dc_shift0_input=off, dc_cycle1=0, dc_cycle1_factor=1, dc_shift1=25000, dc_shift1_factor=0, sdo_01=off, sdo_02=off, sdo_03=on, sdo_04=on, sdo_05=10}
      mask prompts: index "Slave Index"; model "Device Model"; tsample "Sample Time (-1 inherited)"; dc_mode "Mode"; dc_assign_activate "Assign Activate"; dc_cycle0 "Cycle Time Sync 0"; dc_cycle0_factor "Factor"; dc_shift0 "Shift Time Sync0"; dc_shift0_factor "Factor"; dc_shift0_input "Shift Time0 Input"; dc_cycle1 "Cycle Time Sync1"; dc_cycle1_factor "Factor"; dc_shift1 "Shift Time Sync1"; dc_shift1_factor "Factor"; sdo_01 "8000:01 - Enable C reset"; sdo_02 "8000:0E - Reversion of rotation"; sdo_03 "8001:01 - Frequency error counter"; sdo_04 "8001:02 - Amplitude error counter"; sdo_05 "8001:11 - Analog resolution"
      mask help: Beckhoff EtherCAT 1Ch. Sin/Cos Encoder
      mask init:
      | Address = EtherCATSlave.formatAddress(master,index,tsample);
      | 
      | rv = el5021(model).configure(...
      |     [dc_mode, dc_assign_activate, ...
      |     dc_cycle0, dc_cycle0_factor,...
      |     dc_shift0, dc_shift0_factor, dc_shift0_input,...
      |     dc_cycle1, dc_cycle1_factor,...
      |     dc_shift1, dc_shift1_factor], ...
      |     [sdo_01, sdo_02, sdo_03, sdo_04, sdo_05]);
      |  
      | rv.PortConfig.swap_io = EtherCATSlave.shouldSwapIoPorts();
      | 
      | EtherCATSlave.setPortNames(...
      |     {rv.PortConfig.input.portname},...
      |     {rv.PortConfig.output.portname});
      | 
      | set_param(gcb,'AttributesFormatString',...
      |     sprintf('%s\nM:%i Idx:%s',...
      |             model,master,mat2str(index)))
  EL5101_0 : S-Function  LoadFcn=|  FunctionName=ec_slave3  Parameters=Address,rv.SlaveConfig,rv.PortConfig,debug,tsample  SFunctionModules='ecrt_support'  EnableBusSupport=off  mask(EL5101){master=0, index=1, model=EL5101, dcmode=FreeRun/SM-Synchron, x1601=off, x1602=off, x1603=on, x1A01=off, x1A02=off, x1A03=on, x1A04=off, x1A05=off, x1A06=off, x1A07=off, x1A08=off, tsample=0, debug=0, n8000_01=off, n8000_02=off, n8000_03=off, n8000_04=on, n8000_05=off, n8001_01=100, n8001_02=65535, x8010_01=off, x8010_02=off, x8010_03=off, x8010_04=Enable pos. gate, x8010_08=on, x8010_0A=off, x8010_0B=on, x8010_0C=on, x8010_0D=off, x8010_0E=off, x8010_10=on, x8010_11=10000, x8010_13=100, x8010_14=100, x8010_15=100, x8010_16=500, x8010_17=1600}
      | el5101('check')
      | if ~strcmp(bdroot(gcb),'etherlab_lib')
      |   disp([gcb ' is obsolete. Please replace'])
      | end
      mask prompts: index "Slave Index"; model "Device Model"; dcmode "DC Mode"; x1601 "RxPdo #x1601 (Excl 1602,1603)"; x1602 "RxPdo #x1602 (Excl 1601,1603)"; x1603 "RxPdo #x1603 (Excl 1601,1602)"; x1A01 "TxPdo #x1a01 (Excl 1a03,1a04,1a05,1a06,1a07,1a08)"; x1A02 "TxPdo #x1a02 (Excl 1a03,1a04,1a05,1a06,1a07,1a08)"; x1A03 "TxPdo #x1a03 (Excl 1a01,1a02,1a04)"; x1A04 "TxPdo #x1a04 (Excl 1a01,1a02,1a03)"; x1A05 "TxPdo #x1a05 (Excl 1a01,1a02,1a06)"; x1A06 "TxPdo #x1a06 (Excl 1a01,1a02,1a05)"; x1A07 "TxPdo #x1a07 (Excl 1a01,1a02,1a08)"; x1A08 "TxPdo #x1a08 (Excl 1a01,1a02,1a07)"; tsample "Sample Time (-1 inherited)"; n8000_01 "8000:01 - Enable Register Reload"; n8000_02 "8000:02 - Enable Index Reset"; n8000_03 "8000:03 - Enable FWD Count"; n8000_04 "8000:04 - Enable Positive Gate"; n8000_05 "8000:05 - Enable Negaitive Gate"; n8001_01 "8001:01 - Frequency Window"; n8001_02 "8001:02 - Counter Reload Value"; x8010_01 "8010:01 - Enable C reset"; x8010_02 "8010:02 - Enable extern reset"; x8010_03 "8010:03 - Enable up/down counter"; x8010_04 "8010:04 - Gate polarity"; x8010_08 "8010:08 - Disable filter"; x8010_0A "8010:0A - Enable micro increments"; x8010_0B "8010:0B - Open cct det A"; x8010_0C "8010:0C - Open cct det B"; x8010_0D "8010:0D - Open cct det C"; x8010_0E "8010:0E - Reversion of rotation"; x8010_10 "8010:10 - Extern Reset polarity"; x8010_11 "8010:11 - Frequency window"; x8010_13 "8010:13 - Frequency scaling"; x8010_14 "8010:14 - Period scaling"; x8010_15 "8010:15 - Frequency resolution"; x8010_16 "8010:16 - Period resolution"; x8010_17 "8010:17 - Frequency Wait Time"
      mask help: Beckhoff EtherCAT Incremental Encoder Input
      mask init:
      | Address = EtherCATSlave.formatAddress(master,index,tsample);
      | 
      | el5101('set');
      | rv = get_param(gcbh,'UserData');
      | rv.SlaveConfig.sdo = {...
      |     hex2dec('1011'), 1,32,hex2dec('64616f6c');
      |     hex2dec('8000'), 1, 8,n8000_01;
      |     hex2dec('8000'), 2, 8,n8000_02;
      |     hex2dec('8000'), 3, 8,n8000_03;
      |     hex2dec('8000'), 4, 8,n8000_04;
      |     hex2dec('8000'), 5, 8,n8000_05;
      |     hex2dec('8001'), 1,16,n8001_01;
      |     hex2dec('8001'), 2,16,n8001_02;
      |     hex2dec('8010'), 1, 8,x8010_01;
      |     hex2dec('8010'), 2, 8,x8010_02;
      |     hex2dec('8010'), 3, 8,x8010_03;
      |     hex2dec('8010'), 4, 8,x8010_04-1;
      |     hex2dec('8010'), 8, 8,x8010_08;
      |     hex2dec('8010'),10, 8,x8010_0A;
      |     hex2dec('8010'),11, 8,x8010_0B;
      |     hex2dec('8010'),12, 8,x8010_0C;
      |     hex2dec('8010'),13, 8,x8010_0D;
      |     hex2dec('8010'),14, 8,x8010_0E;
      |     hex2dec('8010'),16, 8,x8010_10;
      |     hex2dec('8010'),17,16,x8010_11;
      |     hex2dec('8010'),19,16,x8010_13;
      |     hex2dec('8010'),20,16,x8010_14;
      |     hex2dec('8010'),21,16,x8010_15;
      |     hex2dec('8010'),22,16,x8010_16;
      |     hex2dec('8010'),23,16,x8010_17;
      | };
      | rv.PortConfig.swap_io = EtherCATSlave.shouldSwapIoPorts();
  EL5101_0010_0 : S-Function  LoadFcn=|  FunctionName=ec_slave3  Parameters=Address,rv.SlaveConfig,rv.PortConfig,debug,tsample  SFunctionModules='ecrt_support'  EnableBusSupport=off  mask(EL5101-0010){master=0, index=1, model=EL5101-0010, dcmode=FreeRun/SM-Synchron, x1600=on, x1601=off, x1A00=on, x1A01=off, x1A02=off, x1A03=off, x1A04=off, x1A05=off, tsample=0, debug=0, x8000_01=off, x8000_02=off, x8000_04=Enable pos. gate, x8000_0B=on, x8000_0C=on, x8000_0D=off, x8000_0E=off, x8000_10=on, x8000_11=10000, x8000_13=100, x8000_14=100, x8000_15=100, x8000_16=100, x8000_17=400}
      | el5101_0010('check')
      | if ~strcmp(bdroot(gcb),'etherlab_lib')
      |   disp([gcb ' is obsolete. Please replace'])
      | end
      mask prompts: index "Slave Index"; model "Device Model"; dcmode "DC Mode"; x1600 "RxPdo #x1600 (Excl 1601)"; x1601 "RxPdo #x1601 (Excl 1600)"; x1A00 "TxPdo #x1a00 (Excl 1a01)"; x1A01 "TxPdo #x1a01 (Excl 1a00)"; x1A02 "TxPdo #x1a02 (Excl 1a03)"; x1A03 "TxPdo #x1a03 (Excl 1a02)"; x1A04 "TxPdo #x1a04 (Excl 1a05)"; x1A05 "TxPdo #x1a05 (Excl 1a04)"; tsample "Sample Time (-1 inherited)"; x8000_01 "8000:01 - Enable C reset"; x8000_02 "8000:02 - Enable extern reset"; x8000_04 "8000:04 - Gate polarity"; x8000_0B "8000:0B - Open cct det A"; x8000_0C "8000:0C - Open cct det B"; x8000_0D "8000:0D - Open cct det C"; x8000_0E "8000:0E - Reversion of rotation"; x8000_10 "8000:10 - Extern Reset polarity"; x8000_11 "8000:11 - Frequency window"; x8000_13 "8000:13 - Frequency scaling"; x8000_14 "8000:14 - Period scaling"; x8000_15 "8000:15 - Frequency resolution"; x8000_16 "8000:16 - Period resolution"; x8000_17 "8000:17 - Frequency Wait Time"
      mask help: Beckhoff EtherCAT Incremental Encoder Input
      mask init:
      | Address = EtherCATSlave.formatAddress(master,index,tsample);
      | 
      | el5101_0010('set');
      | rv = get_param(gcbh,'UserData');
      | rv.SlaveConfig.sdo = {...
      |     hex2dec('1011'), 1,32,hex2dec('64616f6c');
      |     hex2dec('8000'), 1, 8,x8000_01;
      |     hex2dec('8000'), 2, 8,x8000_02;
      |     hex2dec('8000'), 4, 8,x8000_04-1;
      |     hex2dec('8000'),11, 8,x8000_0B;
      |     hex2dec('8000'),12, 8,x8000_0C;
      |     hex2dec('8000'),13, 8,x8000_0D;
      |     hex2dec('8000'),14, 8,x8000_0E;
      |     hex2dec('8000'),16, 8,x8000_10;
      |     hex2dec('8000'),17,16,x8000_11;
      |     hex2dec('8000'),19,16,x8000_13;
      |     hex2dec('8000'),20,16,x8000_14;
      |     hex2dec('8000'),21,16,x8000_15;
      |     hex2dec('8000'),22,16,x8000_16;
      |     hex2dec('8000'),23,16,x8000_17;
      | };
      | 
      | rv.PortConfig.swap_io = EtherCATSlave.shouldSwapIoPorts();
  EL515x_1 : S-Function  LoadFcn=|  FunctionName=ec_slave3  Parameters=Address,rv.SlaveConfig,rv.PortConfig,debug,tsample  SFunctionModules='ecrt_support'  EnableBusSupport=off  mask(EL515x){master=0, index=1, model=EL5152, dcmode=FreeRun/SM-Synchron, x1600=on, x1601=off, x1602=off, x1603=off, x1A00=on, x1A01=off, x1A02=off, x1A03=off, x1A04=off, x1A05=off, x1A06=off, x1A07=off, tsample=0, debug=0, x8000_01=off, x8000_02=off, x8000_03=off, x8000_04=Enable pos. gate, x8000_08=off, x8000_0A=off, x8000_0E=off, x8000_0F=off, x8000_10=on, x8000_11=10000, x8000_13=100, x8000_14=100, x8000_15=100, x8000_16=100, x8000_17=1600, x8010_03=off, x8010_08=off, x8010_0A=off, x8010_0E=off, x8010_0F=off, x8010_11=10000, x8010_13=100, x8010_14=100, x8010_15=100, x8010_16=100, x8010_17=1600}
      | el515x('check')
      | if ~strcmp(bdroot(gcb),'etherlab_lib')
      |   disp([gcb ' is obsolete. Please replace'])
      | end
      mask prompts: index "Slave Index"; model "Device Model"; dcmode "DC Mode"; x1600 "RxPdo #x1600 (Excl 1601)"; x1601 "RxPdo #x1601 (Excl 1600)"; x1602 "RxPdo #x1602 (Excl 1603)"; x1603 "RxPdo #x1603 (Excl 1602)"; x1A00 "TxPdo #x1a00 (Excl 1a01)"; x1A01 "TxPdo #x1a01 (Excl 1a00)"; x1A02 "TxPdo #x1a02 (Excl 1a03)"; x1A03 "TxPdo #x1a03 (Excl 1a02)"; x1A04 "TxPdo #x1a04 (Excl 1a05)"; x1A05 "TxPdo #x1a05 (Excl 1a04)"; x1A06 "TxPdo #x1a06 (Excl 1a07)"; x1A07 "TxPdo #x1a07 (Excl 1a06)"; tsample "Sample Time (-1 inherited)"; x8000_01 "8000:01 - Enable C reset"; x8000_02 "8000:02 - Enable extern reset"; x8000_03 "8000:03 - Enable up/down counter"; x8000_04 "8000:04 - Gate polarity"; x8000_08 "8000:08 - Disable filter"; x8000_0A "8000:0A - Enable micro increments"; x8000_0E "8000:0E - Reversion of rotation"; x8000_0F "8000:0F - Freqency window in ms"; x8000_10 "8000:10 - Extern Reset polarity"; x8000_11 "8000:11 - Frequency window"; x8000_13 "8000:13 - Frequency scaling"; x8000_14 "8000:14 - Period scaling"; x8000_15 "8000:15 - Frequency resolution"; x8000_16 "8000:16 - Period resolution"; x8000_17 "8000:17 - Frequency Wait Time"; x8010_03 "8010:03 - Enable up/down counter"; x8010_08 "8010:08 - Disable filter"; x8010_0A "8010:0A - Enable micro increments"; x8010_0E "8010:0E - Reversion of rotation"; x8010_0F "8010:0F - Freqency window in ms"; x8010_11 "8010:11 - Frequency window"; x8010_13 "8010:13 - Frequency scaling"; x8010_14 "8010:14 - Period scaling"; x8010_15 "8010:15 - Frequency resolution"; x8010_16 "8010:16 - Period resolution"; x8010_17 "8010:17 - Frequency Wait Time"
      mask help: Beckhoff EtherCAT Incremental Encoder Input
      mask init:
      | Address = EtherCATSlave.formatAddress(master,index,tsample);
      | 
      | el515x('set');
      | rv = get_param(gcbh,'UserData');
      | rv.SlaveConfig.sdo = {...
      |     hex2dec('8000'), 3, 8,x8000_03;
      |     hex2dec('8000'), 8, 8,x8000_08;
      |     hex2dec('8000'),10, 8,x8000_0A;
      |     hex2dec('8000'),14, 8,x8000_0E;
      |     hex2dec('8000'),15, 8,x8000_0F;
      |     hex2dec('8000'),17,16,x8000_11;
      |     hex2dec('8000'),19,16,x8000_13;
      |     hex2dec('8000'),20,16,x8000_14;
      |     hex2dec('8000'),21,16,x8000_15;
      |     hex2dec('8000'),22,16,x8000_16;
      |     hex2dec('8000'),23,16,x8000_17;
      | };
      | 
      | if strncmp(model,'EL5151',6)
      |     rv.SlaveConfig.sdo = vertcat(rv.SlaveConfig.sdo,...
      |         { hex2dec('8000'), 1, 8,x8000_01;
      |           hex2dec('8000'), 2, 8,x8000_02;
      |           hex2dec('8000'), 4, 8,x8000_04;
      |           hex2dec('8000'),16, 8,x8000_10});
      | else
      |     rv.SlaveConfig.sdo = vertcat(rv.SlaveConfig.sdo,...
      |         { hex2dec('8010'), 3, 8,x8010_03;
      |           hex2dec('8010'), 8, 8,x8010_08;
      |           hex2dec('8010'),10, 8,x8010_0A;
      |           hex2dec('8010'),14, 8,x8010_0E;
      |           hex2dec('8010'),15, 8,x8010_0F;
      |           hex2dec('8010'),17,16,x8010_11;
      |           hex2dec('8010'),19,16,x8010_13;
      |           hex2dec('8010'),20,16,x8010_14;
      |           hex2dec('8010'),21,16,x8010_15;
      |           hex2dec('8010'),22,16,x8010_16;
      |           hex2dec('8010'),23,16,x8010_17});
      | end
      | 
      | rv.PortConfig.swap_io = EtherCATSlave.shouldSwapIoPorts();
  EL51xx_0 : S-Function  LoadFcn=el51xx().checkModelName()  FunctionName=ec_slave3  Parameters=Address,rv.SlaveConfig,rv.PortConfig,debug,tsample  SFunctionModules='ecrt_support'  EnableBusSupport=off  mask(EL51xx){master=0, index=1, model=EL5101, revision=, pdo_x1600=off, pdo_x1601=on, pdo_x1602=off, pdo_x1603=off, pdo_x1A00=off, pdo_x1A01=on, pdo_x1A02=off, pdo_x1A03=off, pdo_x1A04=off, pdo_x1A05=off, pdo_x1A06=off, pdo_x1A07=off, tsample=-1, debug=0, dc_mode=FreeRun/SM-Synchron, dc_assign_activate=hex2dec('320')    % EL51x1: '320'; El5152: '720', dc_cycle0=0, dc_cycle0_factor=1, dc_shift0=0, dc_shift0_factor=0, dc_shift0_input=off, dc_cycle1=0, dc_cycle1_factor=1, dc_shift1=0, dc_shift1_factor=0, sdo_01=off, sdo_02=off, sdo_03=off, sdo_04=on, sdo_05=off, sdo_06=off, sdo_07=off, sdo_08=off, sdo_09=Enable pos. gate, sdo_10=off, sdo_11=off, sdo_12=on, sdo_13=on, sdo_14=off, sdo_15=off, sdo_16=us, sdo_17=Rising edge, sdo_18=10000, sdo_19=100, sdo_20=100, sdo_21=100, sdo_22=100, sdo_23=1600, sdo_24=100, sdo_25=65535, sdo_26=off, sdo_27=off, sdo_28=off, sdo_29=Enable pos. gate, sdo_30=off, sdo_31=off, sdo_32=on, sdo_33=on, sdo_34=off, sdo_35=off, sdo_36=us, sdo_37=Rising edge, sdo_38=10000, sdo_39=100, sdo_40=100, sdo_41=100, sdo_42=100, sdo_43=1600}
      mask prompts: index "Slave Index"; model "Device Model"; pdo_x1600 "RxPdo #x1600"; pdo_x1601 "RxPdo #x1601"; pdo_x1602 "RxPdo #x1602"; pdo_x1603 "RxPdo #x1603"; pdo_x1A00 "TxPdo #x1a00"; pdo_x1A01 "TxPdo #x1a01"; pdo_x1A02 "TxPdo #x1a02"; pdo_x1A03 "TxPdo #x1a03"; pdo_x1A04 "TxPdo #x1a04"; pdo_x1A05 "TxPdo #x1a05"; pdo_x1A06 "TxPdo #x1a06"; pdo_x1A07 "TxPdo #x1a07"; tsample "Sample Time (-1 inherited)"; dc_mode "DC Mode"; dc_assign_activate "Assign Activate"; dc_cycle0 "Cycle Time Sync 0 [ns]"; dc_cycle0_factor "Factor"; dc_shift0 "Shift Time Sync0 [ns]"; dc_shift0_factor "Factor"; dc_shift0_input "Shift Time0 Input"; dc_cycle1 "Cycle Time Sync1 [ns]"; dc_cycle1_factor "Factor"; dc_shift1 "Shift Time Sync1 [ns]"; dc_shift1_factor "Factor"; sdo_01 "8000:01 - Enable register reload"; sdo_02 "8000:02 - Enable index reset"; sdo_03 "8000:03 - Enable FWD count"; sdo_04 "8000:04 - Enable pos. gate"; sdo_05 "8000:05 - Enable neg. gate"; sdo_06 "8000:01 - Enable C reset"; sdo_07 "8000:02 - Enable extern reset"; sdo_08 "8000:03 - Enable up/down counter"; sdo_09 "8000:04 - Gate polarity"; sdo_10 "8000:08 - Disable filter"; sdo_11 "8000:0A - Enable micro increments"; sdo_12 "8000:0B - Open circuit detection A"; sdo_13 "8000:0C - Open circuit detection B"; sdo_14 "8000:0D - Open circuit detection C"; sdo_15 "8000:0E - Reversion of rotation"; sdo_16 "8000:0F - Frequency window base (8000:11)"; sdo_17 "8000:10 - Extern reset polarity"; sdo_18 "8000:11 - Frequency window"; sdo_19 "8000:13 - Frequency scaling [1/Hz]"; sdo_20 "8000:14 - Period scaling [ns]"; sdo_21 "8000:15 - Frequency resolution [1/Hz]"; sdo_22 "8000:16 - Period resolution [ns]"; sdo_23 "8000:17 - Frequency wait time [ms]"; sdo_24 "8001:01 - Frequency window [16us]"; sdo_25 "8001:02 - Counter reload value"; sdo_26 "8010:01 - Enable C reset"; sdo_27 "8010:02 - Enable extern reset"; sdo_28 "8010:03 - Enable up/down counter"; sdo_29 "8010:04 - Gate polarity"; sdo_30 "8010:08 - Disable filter"; sdo_31 "8010:0A - Enable micro increments"; sdo_32 "8010:0B - Open circuit detection A"; sdo_33 "8010:0C - Open circuit detection B"; sdo_34 "8010:0D - Open circuit detection C"; sdo_35 "8010:0E - Reversion of rotation"; sdo_36 "8010:0F - Frequency window base (8010:11)"; sdo_37 "8010:10 - Extern reset polarity"; sdo_38 "8010:11 - Frequency window"; sdo_39 "8010:13 - Frequency scaling [1/Hz]"; sdo_40 "8010:14 - Period scaling [ns]"; sdo_41 "8010:15 - Frequency resolution [1/Hz]"; sdo_42 "8010:16 - Period resolution [ns]"; sdo_43 "8010:17 - Frequency wait time [ms]"
      mask help: Beckhoff EtherCAT Incremental Encoder Input
      mask init:
      | Address = EtherCATSlave.formatAddress(master,index,tsample);
      | 
      | pdo = hex2dec({'1600', '1601', '1602', '1603',...
      |      '1A00', '1A01', '1A02', '1A03', '1A04', ...
      |      '1A05', '1A06', '1A07'});
      |      
      | rv = el51xx(model).configure(...
      |     pdo(boolean([pdo_x1600, pdo_x1601, pdo_x1602, ...
      |                  pdo_x1603, pdo_x1A00, pdo_x1A01, ...
      |                  pdo_x1A02, pdo_x1A03, pdo_x1A04, ...
      |                  pdo_x1A05, pdo_x1A06, pdo_x1A07])), ...
      |     [  sdo_01,   sdo_02,   sdo_03, sdo_04, sdo_05, sdo_06, sdo_07,... 
      |        sdo_08, sdo_09-1,   sdo_10, sdo_11, sdo_12, sdo_13, sdo_14,...
      |        sdo_15, sdo_16-1, sdo_17-1, sdo_18, sdo_19, sdo_20, sdo_21,...
      |        sdo_22,   sdo_23,   sdo_24, sdo_25, sdo_26, sdo_27, sdo_28,...
      |      sdo_29-1,   sdo_30,   sdo_31, sdo_32, sdo_33, sdo_34, sdo_35,...
      |      sdo_36-1, sdo_37-1,   sdo_38, sdo_39, sdo_40, sdo_41, sdo_42,...
      |        sdo_43],...
      |     [dc_mode, dc_assign_activate, ...
      |      dc_cycle0, dc_cycle0_factor,...
      |      dc_shift0, dc_shift0_factor, dc_shift0_input,...
      |      dc_cycle1, dc_cycle1_factor,...
      |      dc_shift1, dc_shift1_factor]);     
      | 
      | rv.PortConfig.swap_io = EtherCATSlave.shouldSwapIoPorts();
      | 
      | EtherCATSlave.setPortNames(...
      |     {rv.PortConfig.input.portname},...
      |     {rv.PortConfig.output.portname});
      | 
      | set_param(gcb,'AttributesFormatString',...
      |     sprintf('%s\nM:%i Idx:%s',...
      |             model,master,mat2str(index)))
  EL60xx_0 : S-Function  LoadFcn=el60xx().checkModelName  FunctionName=ec_slave3  Parameters=Address,rv.SlaveConfig,rv.PortConfig,debug,tsample  SFunctionModules='ecrt_support'  EnableBusSupport=off  mask(EL60xx){master=0, index=1, model=EL6001, revision=, vector=on, tsample=0, debug=0, ch1_enable=on, sdo_08=9600, sdo_11=9600, sdo_09=8N1, sdo_01=on, sdo_02=off, sdo_03=off, sdo_04=off, sdo_05=on, sdo_06=off, sdo_07=off, sdo_10=864, ch2_enable=on, sdo_19=9600, sdo_22=9600, sdo_20=8N1, sdo_12=on, sdo_13=off, sdo_14=off, sdo_15=off, sdo_16=on, sdo_17=off, sdo_18=off, sdo_21=864}
      mask prompts: index "Slave Index"; model "Device Model"; vector "Vector Outputs"; tsample "Sample Time"; debug "Debug Level"; ch1_enable "Enable Channel 1"; sdo_08 "8000:11 Baudrate"; sdo_11 "8000:1B Custom Baudrate"; sdo_09 "8000:15 Data Frame"; sdo_01 "8000:01 Enable RTS/CTS"; sdo_02 "8000:02Enable XON/XOFF for TX"; sdo_03 "8000:03Enable XON/XOFF for RX"; sdo_04 "8000:04 Send FIFO Data Continuous"; sdo_05 "8000:05 Transfer Rate Optimization"; sdo_06 "8000:06 Half Duplex"; sdo_07 "8000:07 RS422 Point to Point"; sdo_10 "8000:1A RX Buffer Full Notification Threshold"; ch2_enable "Enable Channel 2"; sdo_19 "8010:11 Baudrate"; sdo_22 "8010:1B Custom Baudrate"; sdo_20 "8010:15 Data Frame"; sdo_12 "8010:01 Enable RTS/CTS"; sdo_13 "8010:02Enable XON/XOFF for TX"; sdo_14 "8010:03Enable XON/XOFF for RX"; sdo_15 "8010:04 Send FIFO Data Continuous"; sdo_16 "8010:05 Transfer Rate Optimization"; sdo_17 "8010:06 Half Duplex"; sdo_18 "8010:07 RS422 Point to Point"; sdo_21 "8010:1A RX Buffer Full Notification Threshold"
      mask help: Beckhoff EtherCAT RS232/RS485
      mask init:
      | Address = EtherCATSlave.formatAddress(master,index,tsample);
      | 
      | baud_rate_map = [4, 5, 6, 7, 8, 9, 10, 11];
      | 
      | sdo_08 = baud_rate_map(sdo_08);
      | sdo_19 = baud_rate_map(sdo_19);
      | 
      | 
      | sdos = [...
      |     sdo_01, sdo_02, sdo_03, sdo_04, sdo_05, sdo_06, ...
      |     sdo_07, sdo_08, sdo_09, sdo_10, sdo_11, ...
      |     sdo_12, sdo_13, sdo_14, sdo_15, sdo_16, sdo_17, ...
      |     sdo_18, sdo_19, sdo_20, sdo_21, sdo_22, ...
      | ];
      | 
      | rv = el60xx(model).configure([ch1_enable; ch2_enable], sdos);
      | 
      | 
      | inp = arrayfun(@(x) x.portname, rv.PortConfig.input, 'UniformOutput', false);
      | outp = arrayfun(@(x) x.portname, rv.PortConfig.output, 'UniformOutput', false);
      | 
      | 
      | EtherCATSlave.setPortNames(inp, outp);
      | rv.PortConfig.swap_io = EtherCATSlave.shouldSwapIoPorts();
  EL9xxx_0 : S-Function  LoadFcn=el9xxx().checkModelName()  FunctionName=ec_slave3  Parameters=Address,rv.SlaveConfig,rv.PortConfig,debug,tsample  SFunctionModules='ecrt_support'  EnableBusSupport=off  mask(EL9xxx){master=0, index=1, model=EL9110, revision=, vector=off, tsample=0, debug=0}
      mask prompts: index "Slave Index"; model "Device Model"; vector "Vector Outputs"; tsample "Sample Time"; debug "Debug Level"
      mask help: Beckhoff EtherCAT System Terminals with diagnosis
      mask init:
      | Address = EtherCATSlave.formatAddress(master,index,tsample);
      | 
      | rv = el9xxx(model).configure(vector);
      | 
      | rv.PortConfig.swap_io = EtherCATSlave.shouldSwapIoPorts();
  EP1xxx_0 : S-Function  LoadFcn=ep1xxx().checkModelName()  FunctionName=ec_slave3  Parameters=Address,rv.SlaveConfig,rv.PortConfig,debug,tsample  SFunctionModules='ecrt_support'  EnableBusSupport=off  mask(EP1xxx){master=0, index=1, model=EP1008-0002, revision=, vector=on, tsample=0, debug=0}
      mask prompts: index "Slave Index"; model "Device Model"; vector "Vector Output"; tsample "Sample Time"; debug "Deug Level"
      mask help: Beckhoff EtherCAT Digital Input Fieldbus Box
      mask init:
      | Address = EtherCATSlave.formatAddress(master,index,tsample);
      | 
      | rv = ep1xxx(model).configure(vector);
      | rv.PortConfig.swap_io = EtherCATSlave.shouldSwapIoPorts();
  EP2xxx_0 : S-Function  LoadFcn=ep2xxx().checkModelName()  FunctionName=ec_slave3  Parameters=Address,rv.SlaveConfig,rv.PortConfig,debug,tsample  SFunctionModules='ecrt_support'  EnableBusSupport=off  mask(EP2xxx){master=0, index=1, model=EP2001-1000, revision=, vector=on, tsample=-1, debug=0}
      mask prompts: index "Slave Index"; model "Device Model"; vector "Vector Input"; tsample "Sample Time"; debug "Debug Level"
      mask help: Beckhoff EtherCAT Digital Output Fieldbus Box
      mask init:
      | Address = EtherCATSlave.formatAddress(master,index,tsample);
      | 
      | rv = ep2xxx(model).configure(vector);
      | rv.PortConfig.swap_io = EtherCATSlave.shouldSwapIoPorts();
  EP31xx_0 : S-Function  LoadFcn=|  FunctionName=ec_slave3  Parameters=Address,rv.SlaveConfig,rv.PortConfig,debug,tsample  SFunctionModules='ecrt_support'  EnableBusSupport=off  mask(EP3xxx){master=0, index=1, model=EP3174-0002, type_1=-10...+10 V, type_2=-10...+10 V, type_3=-10...+10 V, type_4=-10...+10 V, dc=FreeRun/SM-Synchron, dccustomer=[1 hex2dec('700') 0 0 0 0 0 0 0], vector=on, raw=off, scale=1, offset=0, tau=1, status=off, tsample=0, debug=0}
      | ep31xx('check')
      | if ~strcmp(bdroot(gcb),'etherlab_lib')
      |   disp([gcb ' is obsolete. Please replace'])
      | end
      mask prompts: index "Slave Index"; model "Device Model"; type_1 "Channel 1 Type"; type_2 "Channel 2 Type"; type_3 "Channel 3 Type"; type_4 "Channel 4 Type"; dc "DC Mode"; dccustomer "Dc Customer"; vector "Vector Ports"; raw "Raw Bits"; scale "Output Scale (empty for none)"; offset "Output Offset (empty for none)"; tau "LPF Time Constant (sec)"; status "Status Output"; tsample "Sample Time (-1 for inherited)"
      mask help: Beckhoff Analog Input 16-Bit Fieldbus Box
      mask init:
      | Address = EtherCATSlave.formatAddress(master,index,tsample);
      | 
      | ep31xx('set');  % Report errors
      | 
      | rv = get_param(gcbh,'UserData');
      | 
      | rv.PortConfig.swap_io = EtherCATSlave.shouldSwapIoPorts();
  EP31xx_1 : S-Function  LoadFcn=|  FunctionName=ec_slave3  Parameters=Address,rv.SlaveConfig,rv.PortConfig,debug,tsample  SFunctionModules='ecrt_support'  EnableBusSupport=off  mask(EP31xx){master=0, index=1, model=EP3182-1002, revision=, type_1=-10...+10 V, type_2=-10...+10 V, type_3=-10...+10 V, type_4=-10...+10 V, filter=Off, vector=on, status=off, gain=[], offset=[], tau=[], tsample=0, debug=0, omega=, dc_mode=FreeRun/SM-Synchron, dc_assign_activate=hex2dec('700'), dc_cycle0=[], dc_cycle0_factor=[], dc_shift0=[], dc_shift0_factor=[], dc_shift0_input=off, dc_cycle1=[], dc_cycle1_factor=[], dc_shift1=[], dc_shift1_factor=[]}
      | ep31xx_1().checkModelName()
      | EtherCATSlave.checkFilter()
      mask prompts: index "Slave Index"; model "Device Model"; type_1 "Channel 1 Type"; type_2 "Channel 2 Type"; type_3 "Channel 3 Type"; type_4 "Channel 4 Type"; vector "Vector Ports"; status "Status Output"; gain "Output Scale (empty for none)"; offset "Output Offset (empty for none)"; tau "LPF time constant (s)"; tsample "Sample Time (-1 for inherited)"; omega "deprecated"; dc_mode "DC Mode"; dc_assign_activate "Assign Activate"; dc_cycle0 "Cycle Time Sync 0"; dc_cycle0_factor "Factor"; dc_shift0 "Shift Time Sync0"; dc_shift0_factor "Factor"; dc_shift0_input "Shift Time0 Input"; dc_cycle1 "Cycle Time Sync1"; dc_cycle1_factor "Factor"; dc_shift1 "Shift Time Sync1"; dc_shift1_factor "Factor"
      mask help: Beckhoff Analog Input 16-Bit Fieldbus Box
      mask init:
      | Address = EtherCATSlave.formatAddress(master,index,tsample);
      | 
      | rv = ep31xx_1(model).configure(status,vector,...
      |     EtherCATSlave.configureScale(2^15,gain,offset,tau),...
      |     [dc_mode, dc_assign_activate, ...
      |      dc_cycle0, dc_cycle0_factor, ...
      |      dc_shift0, dc_shift0_factor, dc_shift0_input, ...
      |      dc_cycle1, dc_cycle1_factor, ...
      |      dc_shift1, dc_shift1_factor], ...
      |      filter, [type_1,type_2,type_3,type_4]);
      | 
      | rv.PortConfig.swap_io = EtherCATSlave.shouldSwapIoPorts();
      | 
      | if isfield(rv.PortConfig,'input')
      |     inputnames = {rv.PortConfig.input.portname};
      | else
      |     inputnames = {};
      | end
      | 
      | if vector || model(6) == '1'
      |     set_param(gcb,'AttributesFormatString','');
      | 
      |     set_param(gcb,'MaskDisplay',...
      |         sprintf('disp(''%s\\nM:%i Idx:%s'')',...
      |         model,master,mat2str(index)))
      | else
      |     EtherCATSlave.setPortNames({},...
      |         {rv.PortConfig.output.portname})
      |     
      |     set_param(gcb,'AttributesFormatString',...
      |         sprintf('%s\nM:%i Idx:%s',...
      |         model,master,mat2str(index)))
      | end
  EP41xx_0 : S-Function  LoadFcn=|  FunctionName=ec_slave3  Parameters=Address,rv.SlaveConfig,rv.PortConfig,debug,tsample  SFunctionModules='ecrt_support'  EnableBusSupport=off  mask(EP41xx){master=0, index=1, model=EP4174-0002, type_1=0...10 V, type_2=0...10 V, type_3=0...10 V, type_4=0...10 V, dcmode=FreeRun/SM-Synchron, dccustom=[hex2dec('730'),0,1,0,0,0,0,1,140000,0], vector=on, scale=, tsample=-1, debug=0}
      | ep41xx('check')
      | if ~strcmp(bdroot(gcb),'etherlab_lib')
      |   disp([gcb ' is obsolete. Please replace'])
      | end
      mask prompts: index "Slave Index"; model "Device Model"; type_1 "Channel 1 Type"; type_2 "Channel 2 Type"; type_3 "Channel 3 Type"; type_4 "Channel 4 Type"; dcmode "DC Mode"; dccustom "DC-Customized"; vector "Vector Input"; scale "Input Scale (empty for none)"; tsample "Sample Time (-1 for inherited)"
      mask help: Beckhoff Analog Output Fieldbus Box
      mask init:
      | Address = EtherCATSlave.formatAddress(master,index,tsample);
      | 
      | ep41xx('set');  % Report errors
      | 
      | rv = get_param(gcbh,'UserData');
      | 
      | basetype = [type_1; type_2; type_3; type_4] - 1;
      | type_eq3 = basetype == 3;
      | basetype = basetype .* ~type_eq3 + type_eq3*6;
      | 
      | rowcount = numel(rv.SlaveConfig.sm{1}{3});
      | 
      | rv.SlaveConfig.sdo = num2cell(horzcat(...
      |     hex2dec('F800')*ones(rowcount,1),...
      |     (1:rowcount)',...
      |     16*ones(rowcount,1),...
      |     basetype));
      | 
      | rv.PortConfig.swap_io = EtherCATSlave.shouldSwapIoPorts();
  EP41xx_1 : S-Function  LoadFcn=ep41xx_1().checkModelName()  FunctionName=ec_slave3  Parameters=Address,rv.SlaveConfig,rv.PortConfig,debug,tsample  SFunctionModules='ecrt_support'  EnableBusSupport=off  mask(EP41xx){master=0, index=1, model=EP4174-0002, revision=, type_1=0...10 V, type_2=0...10 V, type_3=0...10 V, type_4=0...10 V, vector=on, gain=[], tsample=-1, debug=0, dc_mode=FreeRun/SM-Synchron, dc_assign_activate=hex2dec('730'), dc_cycle0=0, dc_cycle0_factor=1, dc_shift0=0, dc_shift0_factor=0, dc_shift0_input=off, dc_cycle1=0, dc_cycle1_factor=1, dc_shift1=140000, dc_shift1_factor=0}
      mask prompts: index "Slave Index"; model "Device Model"; type_1 "Channel 1 Type"; type_2 "Channel 2 Type"; type_3 "Channel 3 Type"; type_4 "Channel 4 Type"; vector "Vector Input"; gain "Input Scale (empty for none)"; tsample "Sample Time (-1 for inherited)"; dc_mode "DC Mode"; dc_assign_activate "Assign Activate"; dc_cycle0 "Cycle Time Sync 0"; dc_cycle0_factor "Factor"; dc_shift0 "Shift Time Sync0"; dc_shift0_factor "Factor"; dc_shift0_input "Shift Time0 Input"; dc_cycle1 "Cycle Time Sync1"; dc_cycle1_factor "Factor"; dc_shift1 "Shift Time Sync1"; dc_shift1_factor "Factor"
      mask help: Beckhoff Analog Output Fieldbus Box
      mask init:
      | Address = EtherCATSlave.formatAddress(master,index,tsample);
      | 
      | rv = ep41xx_1(model).configure(vector,...
      |     EtherCATSlave.configureScale(2^15,gain),...
      |     [dc_mode, dc_assign_activate, ...
      |      dc_cycle0, dc_cycle0_factor, ...
      |      dc_shift0, dc_shift0_factor, dc_shift0_input, ...
      |      dc_cycle1, dc_cycle1_factor, ...
      |      dc_shift1, dc_shift1_factor], ...
      |      [type_1; type_2; type_3; type_4]);
      | 
      | rv.PortConfig.swap_io = EtherCATSlave.shouldSwapIoPorts();
  EP43xx_0 : S-Function  LoadFcn=|  FunctionName=ec_slave3  Parameters=Address,rv.SlaveConfig,rv.PortConfig,debug,tsample  SFunctionModules='ecrt_support'  EnableBusSupport=off  mask(EP4374){master=0, index=1, model=EP4374-0002, type_1=0...10 V, type_2=0...10 V, type_3=0...10 V, type_4=0...10 V, status=off, vector=on, dcmode=FreeRun/SM-Synchron, dccustom=[hex2dec('700') 0 1 0 0 0 0 1 80000 0], i_scale=[], o_scale=[], o_offset=[], tau=[], force=off, tsample=0, debug=0}
      | ep43xx('check');
      | if ~strcmp(bdroot(gcb),'etherlab_lib')
      |   disp([gcb ' is obsolete. Please replace'])
      | end
      mask prompts: index "Slave Index"; model "Device Model"; type_1 "Input type Ch1"; type_2 "Input type Ch2"; type_3 "Output type Ch3"; type_4 "Output type Ch4"; status "Status Output"; vector "Vector IO"; dcmode "DC Mode"; dccustom "DC Customer"; i_scale "Input Scale"; o_scale "Output Scale"; o_offset "Output Offset"; tau "LPF Time Constant (sec)"; force "IO Force"; tsample "Sample Time (-1 for inherited)"
      mask help: Beckhoff Analog Input/Output 16-Bit Fieldbus Box
      mask init:
      | Address = EtherCATSlave.formatAddress(master,index,tsample);
      | 
      | ep43xx('set');
      | 
      | rv = get_param(gcbh,'UserData');
      | 
      | rowcount = numel(rv.SlaveConfig.sm{1}{3}) ...
      |          + numel(rv.SlaveConfig.sm{2}{3});
      | 
      | rv.SlaveConfig.sdo = num2cell(horzcat(...
      |     hex2dec('F800')*ones(rowcount,1),...
      |     (1:rowcount)',...
      |     16*ones(rowcount,1),...
      |     [type_1; type_2; type_3; type_4] - 1));
      | 
      | rv.PortConfig.swap_io = EtherCATSlave.shouldSwapIoPorts();
  EP43xx_1 : S-Function  LoadFcn=|  FunctionName=ec_slave3  Parameters=Address,rv.SlaveConfig,rv.PortConfig,debug,tsample  SFunctionModules='ecrt_support'  EnableBusSupport=off  mask(EP4374){master=0, index=1, model=EP4374-0002, revision=, vector=on, tsample=-1, debug=0, type_1=0...10 V, type_2=-10...+10 V, filter=Off, status=off, o_gain=[], o_offset=[], tau=[], omega=, type_3=-10...+10 V, type_4=-10...+10 V, i_gain=[], dc_mode=FreeRun/SM-Synchron, dc_assign_activate=hex2dec('700'), dc_cycle0=[], dc_cycle0_factor=[], dc_shift0=[], dc_shift0_factor=[], dc_shift0_input=off, dc_cycle1=[], dc_cycle1_factor=[], dc_shift1=[], dc_shift1_factor=[]}
      | ep43xx_1().checkModelName()
      | EtherCATSlave.checkFilter()
      mask prompts: index "Slave Index"; model "Device Model"; vector "Vector IO"; tsample "Sample Time (-1 for inherited)"; type_1 "Analog Input type Ch1"; type_2 "Analog Input type Ch2"; o_gain "Scale"; o_offset "Offset"; tau "LPF time constant (s)"; omega "deprecated"; type_3 "Analog Output type Ch3"; type_4 "Analog Output type Ch4"; i_gain "Scale"; dc_mode "DC Mode"; dc_assign_activate "Assign Activate"; dc_cycle0 "Cycle Time Sync 0"; dc_cycle0_factor "Factor"; dc_shift0 "Shift Time Sync0"; dc_shift0_factor "Factor"; dc_shift0_input "Shift Time0 Input"; dc_cycle1 "Cycle Time Sync1"; dc_cycle1_factor "Factor"; dc_shift1 "Shift Time Sync1"; dc_shift1_factor "Factor"
      mask help: Beckhoff Analog Input/Output 16-Bit Fieldbus Box
      mask init:
      | Address = EtherCATSlave.formatAddress(master,index,tsample);
      | 
      | rv = ep43xx_1(model).configure(status,vector,...
      |     EtherCATSlave.configureScale(2^15,o_gain,o_offset,tau,'I'),...
      |     EtherCATSlave.configureScale(2^15,i_gain,[],[],'O'),...
      |     [dc_mode, dc_assign_activate, ...
      |      dc_cycle0, dc_cycle0_factor, ...
      |      dc_shift0, dc_shift0_factor, dc_shift0_input, ...
      |      dc_cycle1, dc_cycle1_factor, ...
      |      dc_shift1, dc_shift1_factor],...
      |      filter,[type_1,type_2,type_3,type_4]);
      | 
      | rv.PortConfig.swap_io = EtherCATSlave.shouldSwapIoPorts();
  EP8309_0 : S-Function  LoadFcn=ep8309().checkModelName()  FunctionName=ec_slave3  Parameters=Address,rv.SlaveConfig,rv.PortConfig,debug,tsample  SFunctionModules='ecrt_support'  EnableBusSupport=off  mask(EP8309){master=0, index=1, model=EP8309-1022, revision=, tsample=0, debug=0, digin=on, digout=on, devstat=off, anain=off, gain=[], offset=[], tau=[], sdo_F800_01=0..20 mA, sdo_F800_02=0..20 mA, sdo_8000_15=Off, filter=, tacho=None, sdo_8020_11=1, sdo_8020_12=100, sdo_8020_15=RPM, sdo_8030_11=1, sdo_8030_12=100, sdo_8030_15=RPM, sdo_8031_0B=on, sdo_8031_0C=off, sdo_8031_11=1, sdo_8031_12=100, sdo_8031_15=RPM, anaout=None, gain2=[], sdo_8050_03=off, sdo_8050_04=off, sdo_8050_05=Set to default, sdo_8050_0D=0, sdo_8050_0E=65535, sdo_8050_10=100, sdo_8050_12=250, sdo_8050_13=4, sdo_8050_14=50, sdo_8050_1E=64, sdo_8050_1F=10, sdo_8060_05=Set to default, sdo_8060_13=4, sdo_8060_14=50, sdo_F800_08=0..20 mA}
      mask prompts: index "Slave Index"; model "Device Model"; tsample "Sample Time (-1 inherited)"; digin "Digital Input"; digout "Digital Output"; devstat "Device Status"; anain "Analog Input"; tau "LPF time constant (s)"; sdo_F800_01 "F800:01 - Output type Ch.1"; sdo_F800_02 "F800:02 - Output type Ch.2"; sdo_8000_15 "8000:06/15 - Hardware filter"; filter "deprecated"; tacho "Tacho Input"; sdo_8020_11 "8020:11 - Targets 1"; sdo_8020_12 "8020:12 - Timeout 1"; sdo_8020_15 "8020:15 - Presentation 1"; sdo_8030_11 "8030:11 - Targets 2"; sdo_8030_12 "8030:12 - Timeout 2"; sdo_8030_15 "8030:15 - Presentation 2"; sdo_8031_0B "8031:0B - Error detection"; sdo_8031_0C "8031:0C - Reversion of rotation"; sdo_8031_11 "8031:11 - Targets"; sdo_8031_12 "8031:12 - Timeout"; sdo_8031_15 "8031:15 - Presentation"; anaout "Analog Output"; gain2 "Gain"; sdo_8050_03 "8050:03 - Dithering"; sdo_8050_04 "8050:04 - Invert polarity"; sdo_8050_05 "8050:05 - Watchdog"; sdo_8050_0D "8050:0D - Default output"; sdo_8050_0E "8050:0E - Default output ramp"; sdo_8050_10 "8050:10 - Max Current [%]"; sdo_8050_12 "8050:12 - Kp factor"; sdo_8050_13 "8050:13 - Ki factor"; sdo_8050_14 "8050:14 - Kd factor"; sdo_8050_1E "8050:1E - Dither frequency [Hz]"; sdo_8050_1F "8050:1F - Dither amplitude [%]"; sdo_8060_05 "8060:05 - Watchdog"; sdo_8060_13 "8060:13 - Default output"; sdo_8060_14 "8060:14 - Default output ramp"; sdo_F800_08 "F800:08 - Output type"
      mask help: Beckhoff Multifunctional I/O EtherCAT Box
      mask init:
      | Address = EtherCATSlave.formatAddress(master,index,tsample);
      | 
      | io = [];
      | 
      | if digin
      |     io.digin = 1;
      | end
      | if digout
      |     io.digout = 1;
      | end
      | if devstat
      |     io.devstat = 1;
      | end
      | if anain
      |     io.anain.gain = gain;
      |     io.anain.offset = offset;
      |     io.anain.filter = tau;
      |     io.anain.sdo = [hex2dec('8000'), hex2dec('06'), sdo_8000_15 > 1;
      |                     hex2dec('8000'), hex2dec('15'), sdo_8000_15 - 1;
      |                     hex2dec('F800'), hex2dec('01'), sdo_F800_01;
      |                     hex2dec('F800'), hex2dec('02'), sdo_F800_02];
      | end
      | tachogain = [1,0.1,0.01,1,0.1,0.01,0.001];
      | switch tacho
      |     case 2  % Single shaft mode
      |         io.tacho1.gain = tachogain(sdo_8031_15);
      |         io.tacho1.sdo = [hex2dec('8031'), hex2dec('0B'), sdo_8031_0B;
      |                          hex2dec('8031'), hex2dec('0C'), sdo_8031_0C;
      |                          hex2dec('8031'), hex2dec('11'), sdo_8031_11;
      |                          hex2dec('8031'), hex2dec('12'), sdo_8031_12;
      |                          hex2dec('8031'), hex2dec('15'), sdo_8031_15];
      |     case 3   % dual shaft mode
      |         io.tacho2.gain = [tachogain(sdo_8020_15), tachogain(sdo_8030_15)];
      |         io.tacho2.sdo = [hex2dec('8020'), hex2dec('11'), sdo_8020_11;
      |                          hex2dec('8020'), hex2dec('12'), sdo_8020_12;
      |                          hex2dec('8020'), hex2dec('15'), sdo_8020_15;
      |                          hex2dec('8030'), hex2dec('11'), sdo_8030_11;
      |                          hex2dec('8030'), hex2dec('12'), sdo_8030_12;
      |                          hex2dec('8030'), hex2dec('15'), sdo_8030_15];
      | end
      | switch anaout
      |     case 2  % Current
      |         io.current.gain = gain2;
      |         io.current.sdo = [hex2dec('8060'), hex2dec('05'), sdo_8060_05;
      |                           hex2dec('8060'), hex2dec('13'), sdo_8060_13;
      |                           hex2dec('8060'), hex2dec('14'), sdo_8060_14;
      |                           hex2dec('F800'), hex2dec('08'), sdo_F800_08];
      |     case 3  % PWM
      |         io.pwm.gain = gain2;
      |         io.pwm.sdo = [hex2dec('8050'), hex2dec('03'), sdo_8050_03;
      |                       hex2dec('8050'), hex2dec('04'), sdo_8050_04;
      |                       hex2dec('8050'), hex2dec('05'), sdo_8050_05;
      |                       hex2dec('8050'), hex2dec('0D'), sdo_8050_0D;
      |                       hex2dec('8050'), hex2dec('0E'), sdo_8050_0E;
      |                       hex2dec('8050'), hex2dec('10'), sdo_8050_10;
      |                       hex2dec('8050'), hex2dec('12'), sdo_8050_12;
      |                       hex2dec('8050'), hex2dec('13'), sdo_8050_13;
      |                       hex2dec('8050'), hex2dec('14'), sdo_8050_14;
      |                       hex2dec('8050'), hex2dec('1E'), sdo_8050_1E;
      |                       hex2dec('8050'), hex2dec('1F'), sdo_8050_1F];
      | end
      | 
      | %save ep
      | rv = ep8309(model).configure(io);
      | 
      | rv.PortConfig.swap_io = EtherCATSlave.shouldSwapIoPorts();
      | 
      | EtherCATSlave.setPortNames(...
      |     {rv.PortConfig.input.portname},...
      |     {rv.PortConfig.output.portname});
      | 
      | set_param(gcb,'AttributesFormatString',...
      |     sprintf('%s\nM:%i Idx:%s',...
      |             model,master,mat2str(index)))
  EXx9xx_0 : S-Function  LoadFcn=exx9xx().checkModelName()  FunctionName=ec_slave3  Parameters=Address,rv.SlaveConfig,rv.PortConfig,debug,tsample  SFunctionModules='ecrt_support'  EnableBusSupport=off  mask(EXx9xx){master=0, index=1, model=EL1904, safein=off, safeout=off, vector=on, tsample=-1, revision=, debug=}
      mask prompts: index "Slave Index"; model "Device Model"; safein "Safe inputs"; safeout "Safe outputs"; tsample "Sample Time (-1 for inherited)"
      mask help: Beckhoff EtherCAT SAFE digital input and/or output
      mask init:
      | Address = EtherCATSlave.formatAddress(master,index,tsample);
      | 
      | rv = exx9xx(model).configure(safein, safeout, vector);
      | 
      | rv.PortConfig.swap_io = EtherCATSlave.shouldSwapIoPorts();
      | 
      | EtherCATSlave.setPortNames(...
      |     {rv.PortConfig.input.portname},...
      |     {rv.PortConfig.output.portname});
      | 
      | set_param(gcb,'AttributesFormatString',...
      |     sprintf('%s\nM:%i Idx:%s',...
      |             model,master,mat2str(index)))
  Infrastructure : S-Function  LoadFcn=ekxxxx().checkModelName()  FunctionName=ec_slave3  Parameters=Address,rv.SlaveConfig,rv.PortConfig,debug,tsample  SFunctionModules='ecrt_support'  EnableBusSupport=off  mask(EKxxxx){master=0, index=1, model=EK1100, revision=, vector=off, tsample=0, debug=0}
      mask prompts: index "Slave Index"; model "Device Model"; vector "Vector output"; tsample "Sample Time / Domain"
      mask help: EtherCAT Infrastructure Slaves. Including these slaves (even if they don't have I/Os) will create slave configurations, which will cause them to go into the operational state.
      mask init:
      | Address = EtherCATSlave.formatAddress(master,index,tsample);
      | 
      | rv = ekxxxx(model).configure(vector);
      | 
      | rv.PortConfig.swap_io = EtherCATSlave.shouldSwapIoPorts();
